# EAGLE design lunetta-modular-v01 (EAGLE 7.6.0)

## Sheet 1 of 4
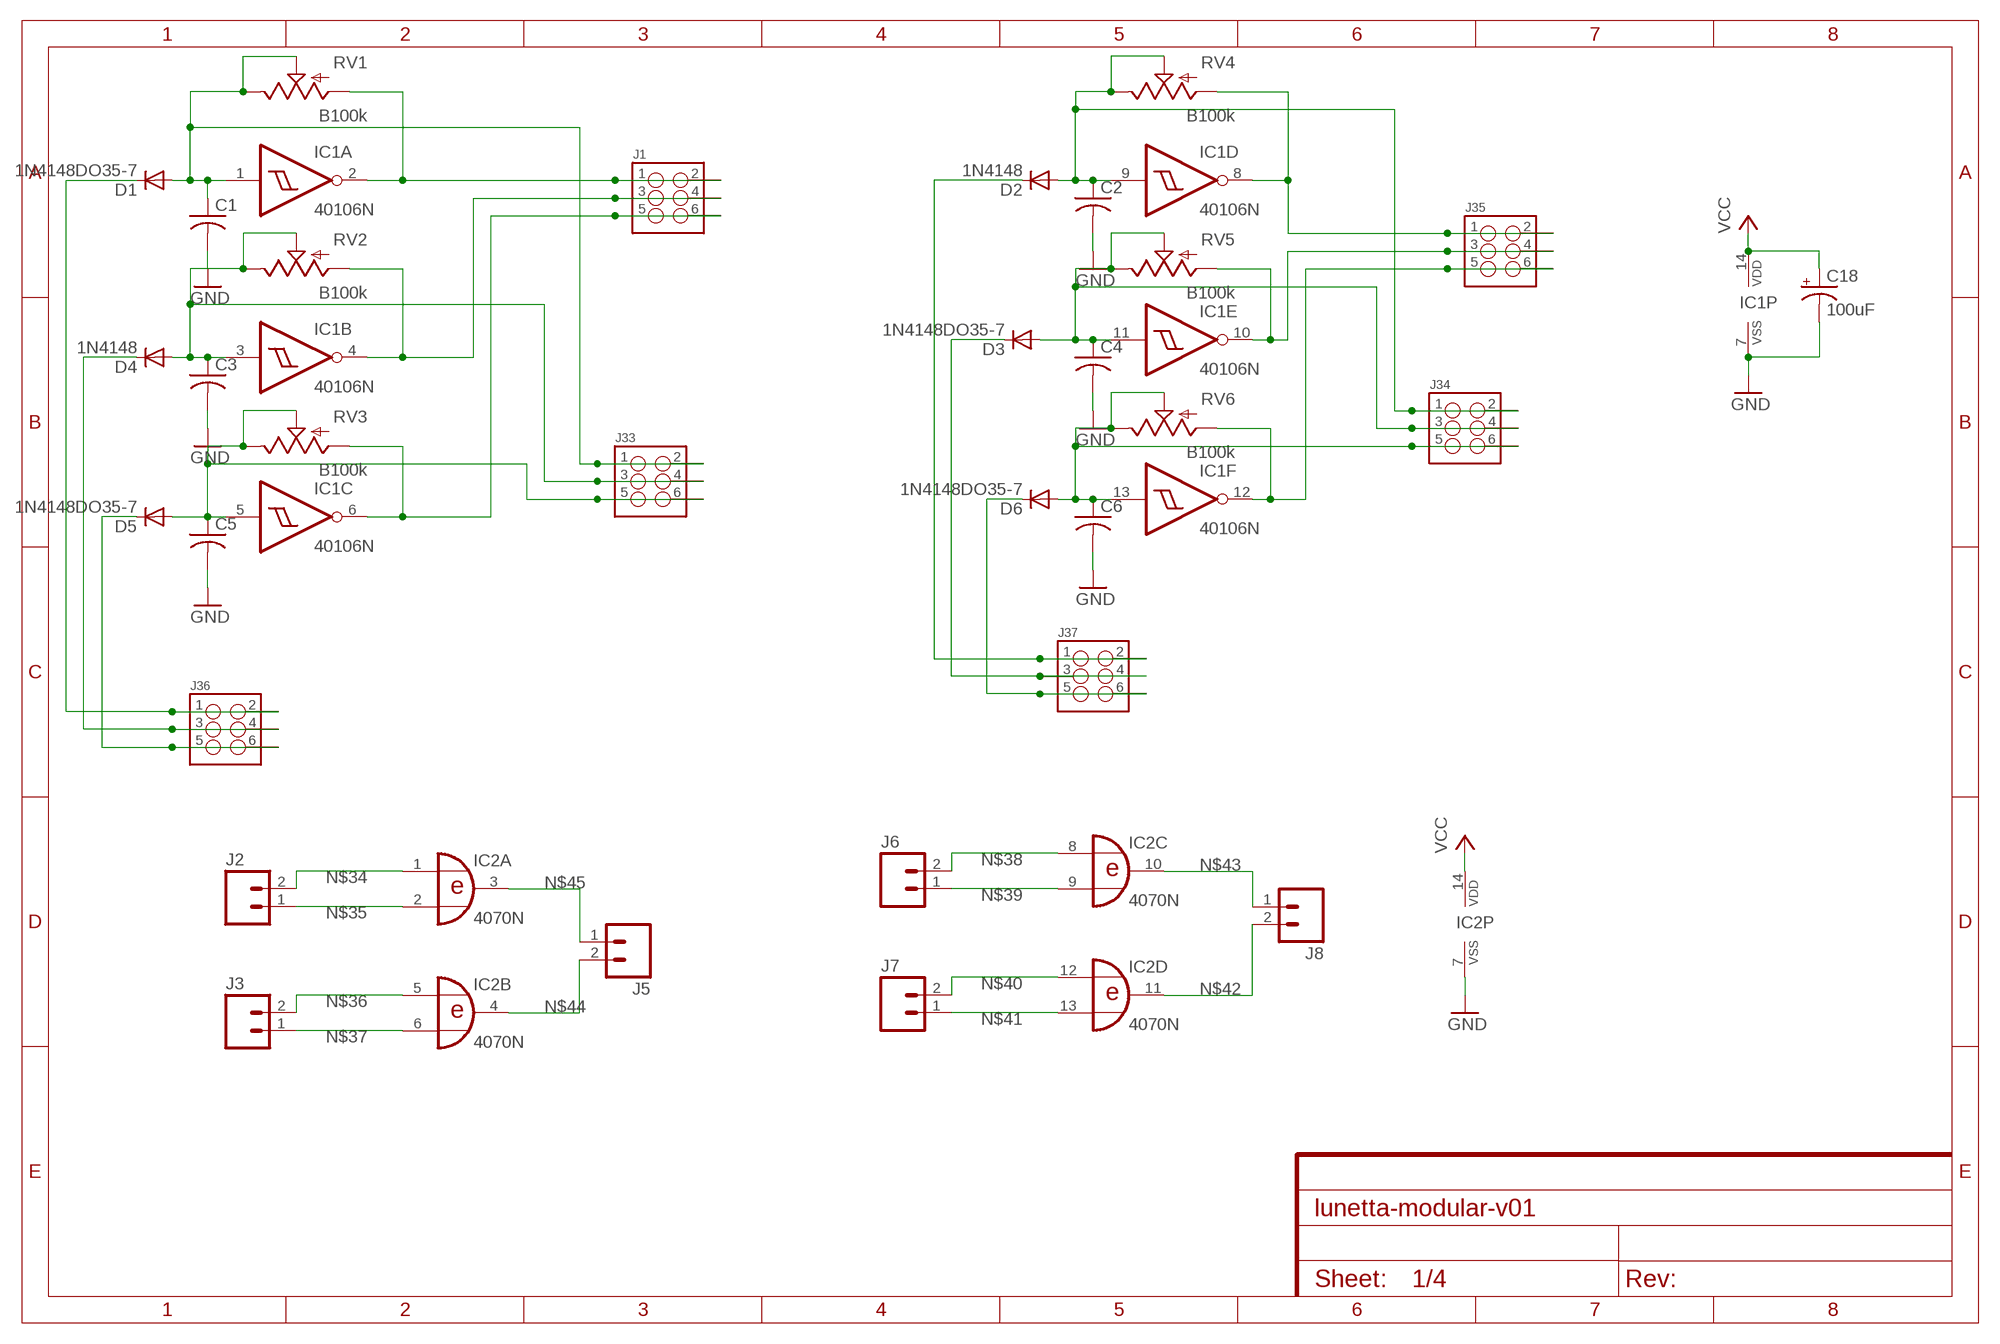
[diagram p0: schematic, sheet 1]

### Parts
C1  C-USC025_050-025X075_2GND  [C025_050-025X075]
C2  C-USC025_050-025X075_2GND  [C025_050-025X075]
C3  C-USC025_050-025X075_2GND  [C025_050-025X075]
C4  C-USC025_050-025X075_2GND  [C025_050-025X075]
C5  C-USC025_050-025X075_2GND  [C025_050-025X075]
C6  C-USC025_050-025X075_2GND  [C025_050-025X075]
C18  100uF  100UF-25V-20%(PTH)  [CPOL-RADIAL-100UF-25V]
D1  1N4148DO35-7  [DO35-7]
D2  1N4148  1N4148DO35-7  [DO35-7]
D3  1N4148DO35-7  [DO35-7]
D4  1N4148  1N4148DO35-7  [DO35-7]
D5  1N4148DO35-7  [DO35-7]
D6  1N4148DO35-7  [DO35-7]
IC1  40106N  [DIL14]
IC2  4070N  [DIL14]
J1  M03X22X3_SILK_MALE_PTH  [2X3]
J2  M02LOCK  [1X02_LOCK]
J3  M02LOCK  [1X02_LOCK]
J5  M02LOCK  [1X02_LOCK]
J6  M02LOCK  [1X02_LOCK]
J7  M02LOCK  [1X02_LOCK]
J8  M02LOCK  [1X02_LOCK]
J33  M03X22X3_SILK_MALE_PTH  [2X3]
J34  M03X22X3_SILK_MALE_PTH  [2X3]
J35  M03X22X3_SILK_MALE_PTH  [2X3]
J36  M03X22X3_SILK_MALE_PTH  [2X3]
J37  M03X22X3_SILK_MALE_PTH  [2X3]
RV1  B100k  POTELCON  [ALPS_POT_ELCON]
RV2  B100k  POTELCON  [ALPS_POT_ELCON]
RV3  B100k  POTELCON  [ALPS_POT_ELCON]
RV4  B100k  POTELCON  [ALPS_POT_ELCON]
RV5  B100k  POTELCON  [ALPS_POT_ELCON]
RV6  B100k  POTELCON  [ALPS_POT_ELCON]

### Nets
GND: C1.2 C1.3 C2.2 C2.3 C3.2 C3.3 C4.2 C4.3 C5.2 C5.3 C6.2 C6.3 C18.2(-) IC1.7(P:VSS) IC2.7(P:VSS) ; also sheet 2,3,4
N$1: D1.C J36.1 J36.2
N$2: D4.C J36.3 J36.4
N$3: D5.C J36.5 J36.6
N$4: D2.C J37.1 J37.2
N$5: D3.C J37.3 J37.4
N$6: D6.C J37.5 J37.6
N$19: IC1.8(D:O) J35.1 J35.2 RV4.P$3(A)
N$31: IC1.4(B:O) J1.3 J1.4 RV2.P$3(A)
N$32: IC1.10(E:O) J35.3 J35.4 RV5.P$3(A)
N$33: IC1.6(C:O) J1.5 J1.6 RV3.P$3(A)
N$34: IC2.1(A:I0) J2.2
N$35: IC2.2(A:I1) J2.1
N$36: IC2.5(B:I0) J3.2
N$37: IC2.6(B:I1) J3.1
N$38: IC2.8(C:I0) J6.2
N$39: IC2.9(C:I1) J6.1
N$40: IC2.12(D:I0) J7.2
N$41: IC2.13(D:I1) J7.1
N$42: IC2.11(D:O) J8.2
N$43: IC2.10(C:O) J8.1
N$44: IC2.4(B:O) J5.2
N$45: IC2.3(A:O) J5.1
N$89: IC1.12(F:O) J35.5 J35.6 RV6.P$3(A)
N$125: IC1.2(A:O) J1.1 J1.2 RV1.P$3(A)
N$127: C1.1 D1.A IC1.1(A:I) J33.1 J33.2 RV1.P$1(E) RV1.P$2(S)
N$131: C3.1 D4.A IC1.3(B:I) J33.3 J33.4 RV2.P$1(E) RV2.P$2(S)
N$144: C5.1 D5.A IC1.5(C:I) J33.5 J33.6 RV3.P$1(E) RV3.P$2(S)
N$145: C2.1 D2.A IC1.9(D:I) J34.1 J34.2 RV4.P$1(E) RV4.P$2(S)
N$146: C4.1 D3.A IC1.11(E:I) J34.3 J34.4 RV5.P$1(E) RV5.P$2(S)
N$147: C6.1 D6.A IC1.13(F:I) J34.5 J34.6 RV6.P$1(E) RV6.P$2(S)
VCC: C18.1(+) IC1.14(P:VDD) IC2.14(P:VDD) ; also sheet 2,3,4

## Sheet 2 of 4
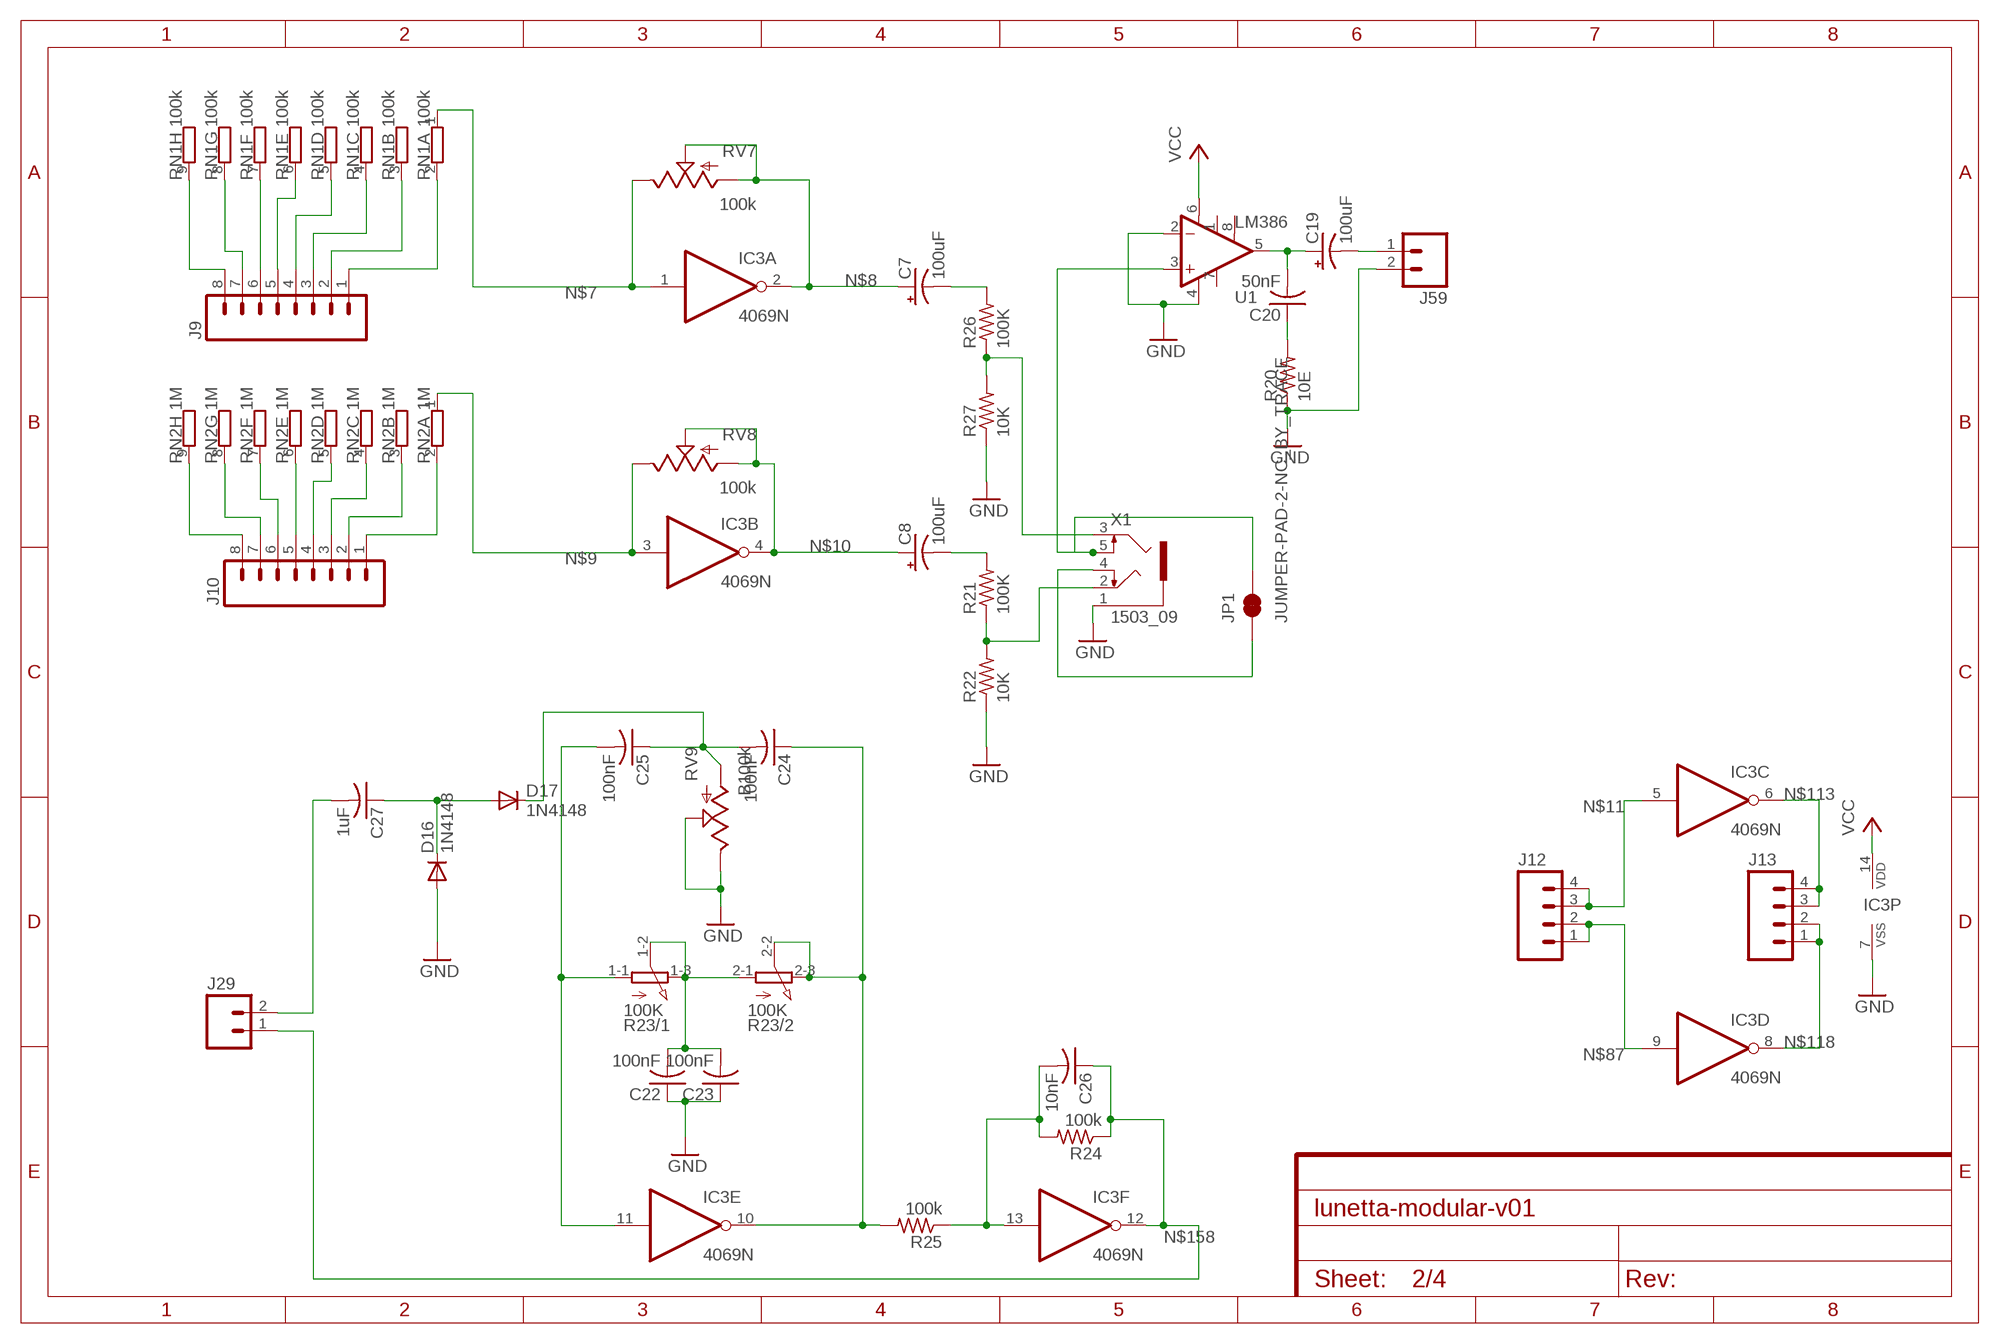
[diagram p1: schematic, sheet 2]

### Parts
C7  100uF  100UF-25V-20%(PTH)  [CPOL-RADIAL-100UF-25V]
C8  100uF  100UF-25V-20%(PTH)  [CPOL-RADIAL-100UF-25V]
C19  100uF  100UF-25V-20%(PTH)  [CPOL-RADIAL-100UF-25V]
C20  50nF  C-US025-025X050  [C025-025X050]
C22  100nF  C-US025-025X050  [C025-025X050]
C23  100nF  C-US025-025X050  [C025-025X050]
C24  100nF  C-US025-025X050  [C025-025X050]
C25  100nF  C-US025-025X050  [C025-025X050]
C26  10nF  C-US025-025X050  [C025-025X050]
C27  1uF  C-US025-025X050  [C025-025X050]
D16  1N4148  1N4148DO35-7  [DO35-7]
D17  1N4148  1N4148DO35-7  [DO35-7]
IC3  4069N  [DIL14]
J9  M08LOCK  [1X08_LOCK]
J10  M08LOCK  [1X08_LOCK]
J12  M042X2  [2X2]
J13  M042X2  [2X2]
J29  M02LOCK  [1X02_LOCK]
J59  M02LOCK  [1X02_LOCK]
JP1  JUMPER-PAD-2-NC_BY_TRACE  [PAD-JUMPER-2-NC_BY_TRACE_YES_SILK]
R20  10E  R-US_0207/10  [0207/10]
R21  100K  R-US_0207/10  [0207/10]
R22  10K  R-US_0207/10  [0207/10]
R23  100K  3RP/1610G  [3RP/1610G]
R24  100k  R-US_0207/10  [0207/10]
R25  100k  R-US_0207/10  [0207/10]
R26  100K  R-US_0207/10  [0207/10]
R27  10K  R-US_0207/10  [0207/10]
RN1  100k  GE08R  [SIL9]
RN2  1M  GE08R  [SIL9]
RV7  100k  POTELCON  [ALPS_POT_ELCON]
RV8  100k  POTELCON  [ALPS_POT_ELCON]
RV9  B100k  POTELCON  [ALPS_POT_ELCON]
U1  LM386  [DIP08]
X1  1503_09  [1503_09]

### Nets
GND: C22.1 C23.1 D16.A IC3.7(P:VSS) J59.2 R20.1 R22.1 R27.1 RV9.P$1(E) RV9.P$2(S) U1.2(-IN) U1.4(V-) X1.1 ; also sheet 1,3,4
N$7: IC3.1(A:I) RN1.1 RV7.P$1(E)
N$8: C7.1(+) IC3.2(A:O) RV7.P$2(S) RV7.P$3(A)
N$9: IC3.3(B:I) RN2.1 RV8.P$1(E)
N$10: C8.1(+) IC3.4(B:O) RV8.P$2(S) RV8.P$3(A)
N$11: IC3.5(C:I) J12.3 J12.4
N$13: JP1.1 X1.4
N$15: C20.1 R20.2
N$16: C19.1(+) C20.2 U1.5(OUT)
N$28: C8.2(-) R21.2
N$87: IC3.9(D:I) J12.1 J12.2
N$88: R26.1 R27.2 X1.3
N$90: C27.2 J29.2
N$92: C26.2 IC3.13(F:I) R24.2 R25.1
N$95: J10.8 RN2.9
N$96: J10.7 RN2.8
N$99: J10.6 RN2.7
N$100: J10.5 RN2.6
N$101: J10.4 RN2.5
N$102: J10.3 RN2.4
N$103: J10.2 RN2.3
N$104: J10.1 RN2.2
N$105: J9.8 RN1.9
N$106: J9.7 RN1.8
N$107: J9.6 RN1.7
N$108: J9.5 RN1.6
N$109: J9.4 RN1.5
N$110: J9.3 RN1.4
N$111: J9.2 RN1.3
N$112: J9.1 RN1.2
N$113: IC3.6(C:O) J13.3 J13.4
N$115: C7.2(-) R26.2
N$118: IC3.8(D:O) J13.1 J13.2
N$130: C19.2(-) J59.1
N$148: R21.1 R22.2 X1.2
N$151: JP1.2 U1.3(+IN) X1.5
N$153: C27.1 D16.C D17.A
N$154: C24.2 C25.1 D17.C RV9.P$3(A)
N$155: C22.2 C23.2 R23.1-2(/1:S) R23.1-3(/1:E) R23.2-1(/2:A)
N$156: C24.1 IC3.10(E:O) R23.2-2(/2:S) R23.2-3(/2:E) R25.2
N$157: C25.2 IC3.11(E:I) R23.1-1(/1:A)
N$158: C26.1 IC3.12(F:O) J29.1 R24.1
VCC: IC3.14(P:VDD) U1.6(V+) ; also sheet 1,3,4
Unconnected: U1.1(GAIN) U1.7(BP) U1.8(GAIN)

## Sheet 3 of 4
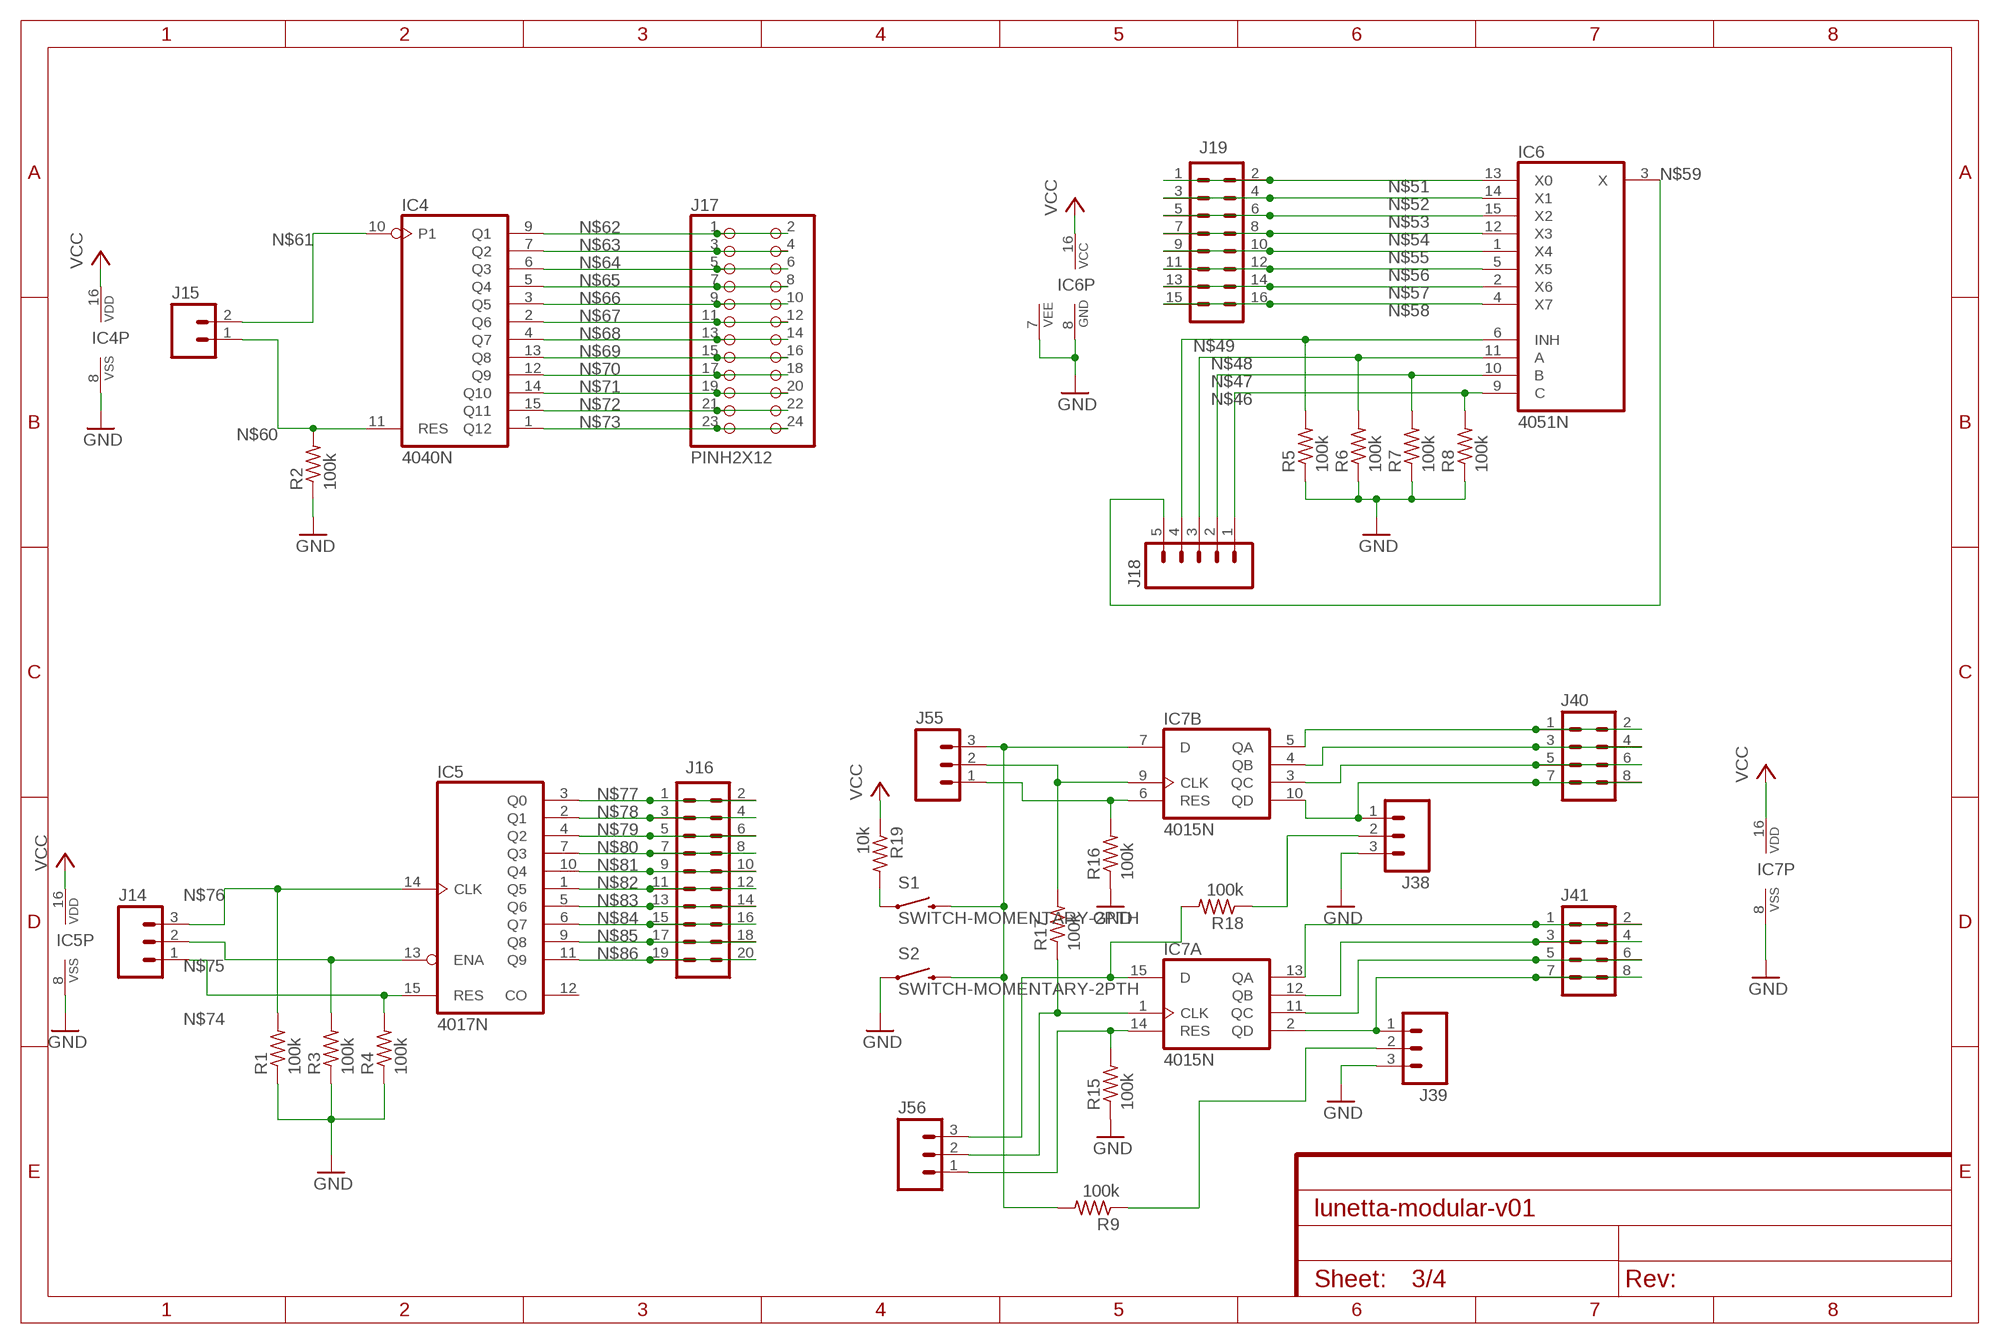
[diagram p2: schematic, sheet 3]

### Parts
IC4  4040N  [DIL16]
IC5  4017N  [DIL16]
IC6  4051N  [DIL16]
IC7  4015N  [DIL16]
J14  M03LOCK  [1X03_LOCK]
J15  M02PTH  [1X02]
J16  M10X2  [2X10]
J17  PINH2X12  [2X12]
J18  M05LOCK  [1X05_LOCK]
J19  M08X2  [2X8]
J38  M03LOCK  [1X03_LOCK]
J39  M03LOCK  [1X03_LOCK]
J40  M04X2  [2X4]
J41  M04X2  [2X4]
J55  M03LOCK  [1X03_LOCK]
J56  M03LOCK  [1X03_LOCK]
R1  100k  R-US_0207/10  [0207/10]
R2  100k  R-US_0207/10  [0207/10]
R3  100k  R-US_0207/10  [0207/10]
R4  100k  R-US_0207/10  [0207/10]
R5  100k  R-US_0207/10  [0207/10]
R6  100k  R-US_0207/10  [0207/10]
R7  100k  R-US_0207/10  [0207/10]
R8  100k  R-US_0207/10  [0207/10]
R9  100k  R-US_0207/10  [0207/10]
R15  100k  R-US_0207/10  [0207/10]
R16  100k  R-US_0207/10  [0207/10]
R17  100k  R-US_0207/10  [0207/10]
R18  100k  R-US_0207/10  [0207/10]
R19  10k  R-US_0207/10  [0207/10]
S1  SWITCH-MOMENTARY-2PTH  [TACTILE-PTH]
S2  SWITCH-MOMENTARY-2PTH  [TACTILE-PTH]

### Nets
GND: IC4.8(VSS) IC5.8(VSS) IC6.7(VEE) IC6.8(GND) IC7.8(P:VSS) J38.3 J39.3 R1.1 R2.1 R3.1 R4.1 R5.1 R6.1 R7.1 R8.1 R15.1 R16.1 S2.1 ; also sheet 1,2,4
N$12: J39.2 R9.1
N$46: IC6.9(C) J18.1 R8.2
N$47: IC6.10(B) J18.2 R7.2
N$48: IC6.11(A) J18.3 R6.2
N$49: IC6.6(INH) J18.4 R5.2
N$51: IC6.13(X0) J19.1 J19.2
N$52: IC6.14(X1) J19.3 J19.4
N$53: IC6.15(X2) J19.5 J19.6
N$54: IC6.12(X3) J19.7 J19.8
N$55: IC6.1(X4) J19.9 J19.10
N$56: IC6.5(X5) J19.11 J19.12
N$57: IC6.2(X6) J19.13 J19.14
N$58: IC6.4(X7) J19.15 J19.16
N$59: IC6.3(X) J18.5
N$60: IC4.11(RES) J15.1 R2.2
N$61: IC4.10(P1) J15.2
N$62: IC4.9(Q1) J17.1 J17.2
N$63: IC4.7(Q2) J17.3 J17.4
N$64: IC4.6(Q3) J17.5 J17.6
N$65: IC4.5(Q4) J17.7 J17.8
N$66: IC4.3(Q5) J17.9 J17.10
N$67: IC4.2(Q6) J17.11 J17.12
N$68: IC4.4(Q7) J17.13 J17.14
N$69: IC4.13(Q8) J17.15 J17.16
N$70: IC4.12(Q9) J17.17 J17.18
N$71: IC4.14(Q10) J17.19 J17.20
N$72: IC4.15(Q11) J17.21 J17.22
N$73: IC4.1(Q12) J17.23 J17.24
N$74: IC5.15(RES) J14.1 R4.2
N$75: IC5.13(ENA) J14.2 R3.2
N$76: IC5.14(CLK) J14.3 R1.2
N$77: IC5.3(Q0) J16.1 J16.2
N$78: IC5.2(Q1) J16.3 J16.4
N$79: IC5.4(Q2) J16.5 J16.6
N$80: IC5.7(Q3) J16.7 J16.8
N$81: IC5.10(Q4) J16.9 J16.10
N$82: IC5.1(Q5) J16.11 J16.12
N$83: IC5.5(Q6) J16.13 J16.14
N$84: IC5.6(Q7) J16.15 J16.16
N$85: IC5.9(Q8) J16.17 J16.18
N$86: IC5.11(Q9) J16.19 J16.20
N$97: IC7.14(A:RES) J56.1 R15.2
N$98: IC7.6(B:RES) J55.1 R16.2
N$124: IC7.9(B:CLK) J55.2 R17.2
N$126: IC7.1(A:CLK) J56.2 R17.1
N$132: IC7.10(B:QD) J38.1 J40.7 J40.8
N$133: IC7.15(A:D) J56.3 R18.2
N$134: J38.2 R18.1
N$135: IC7.2(A:QD) J39.1 J41.7 J41.8
N$136: IC7.7(B:D) J55.3 R9.2 S1.3 S2.3
N$137: R19.2 S1.1
N$138: IC7.11(A:QC) J41.5 J41.6
N$139: IC7.12(A:QB) J41.3 J41.4
N$140: IC7.13(A:QA) J41.1 J41.2
N$141: IC7.3(B:QC) J40.5 J40.6
N$142: IC7.4(B:QB) J40.3 J40.4
N$143: IC7.5(B:QA) J40.1 J40.2
VCC: IC4.16(VDD) IC5.16(VDD) IC6.16(VCC) IC7.16(P:VDD) R19.1 ; also sheet 1,2,4
Unconnected: IC5.12(CO)

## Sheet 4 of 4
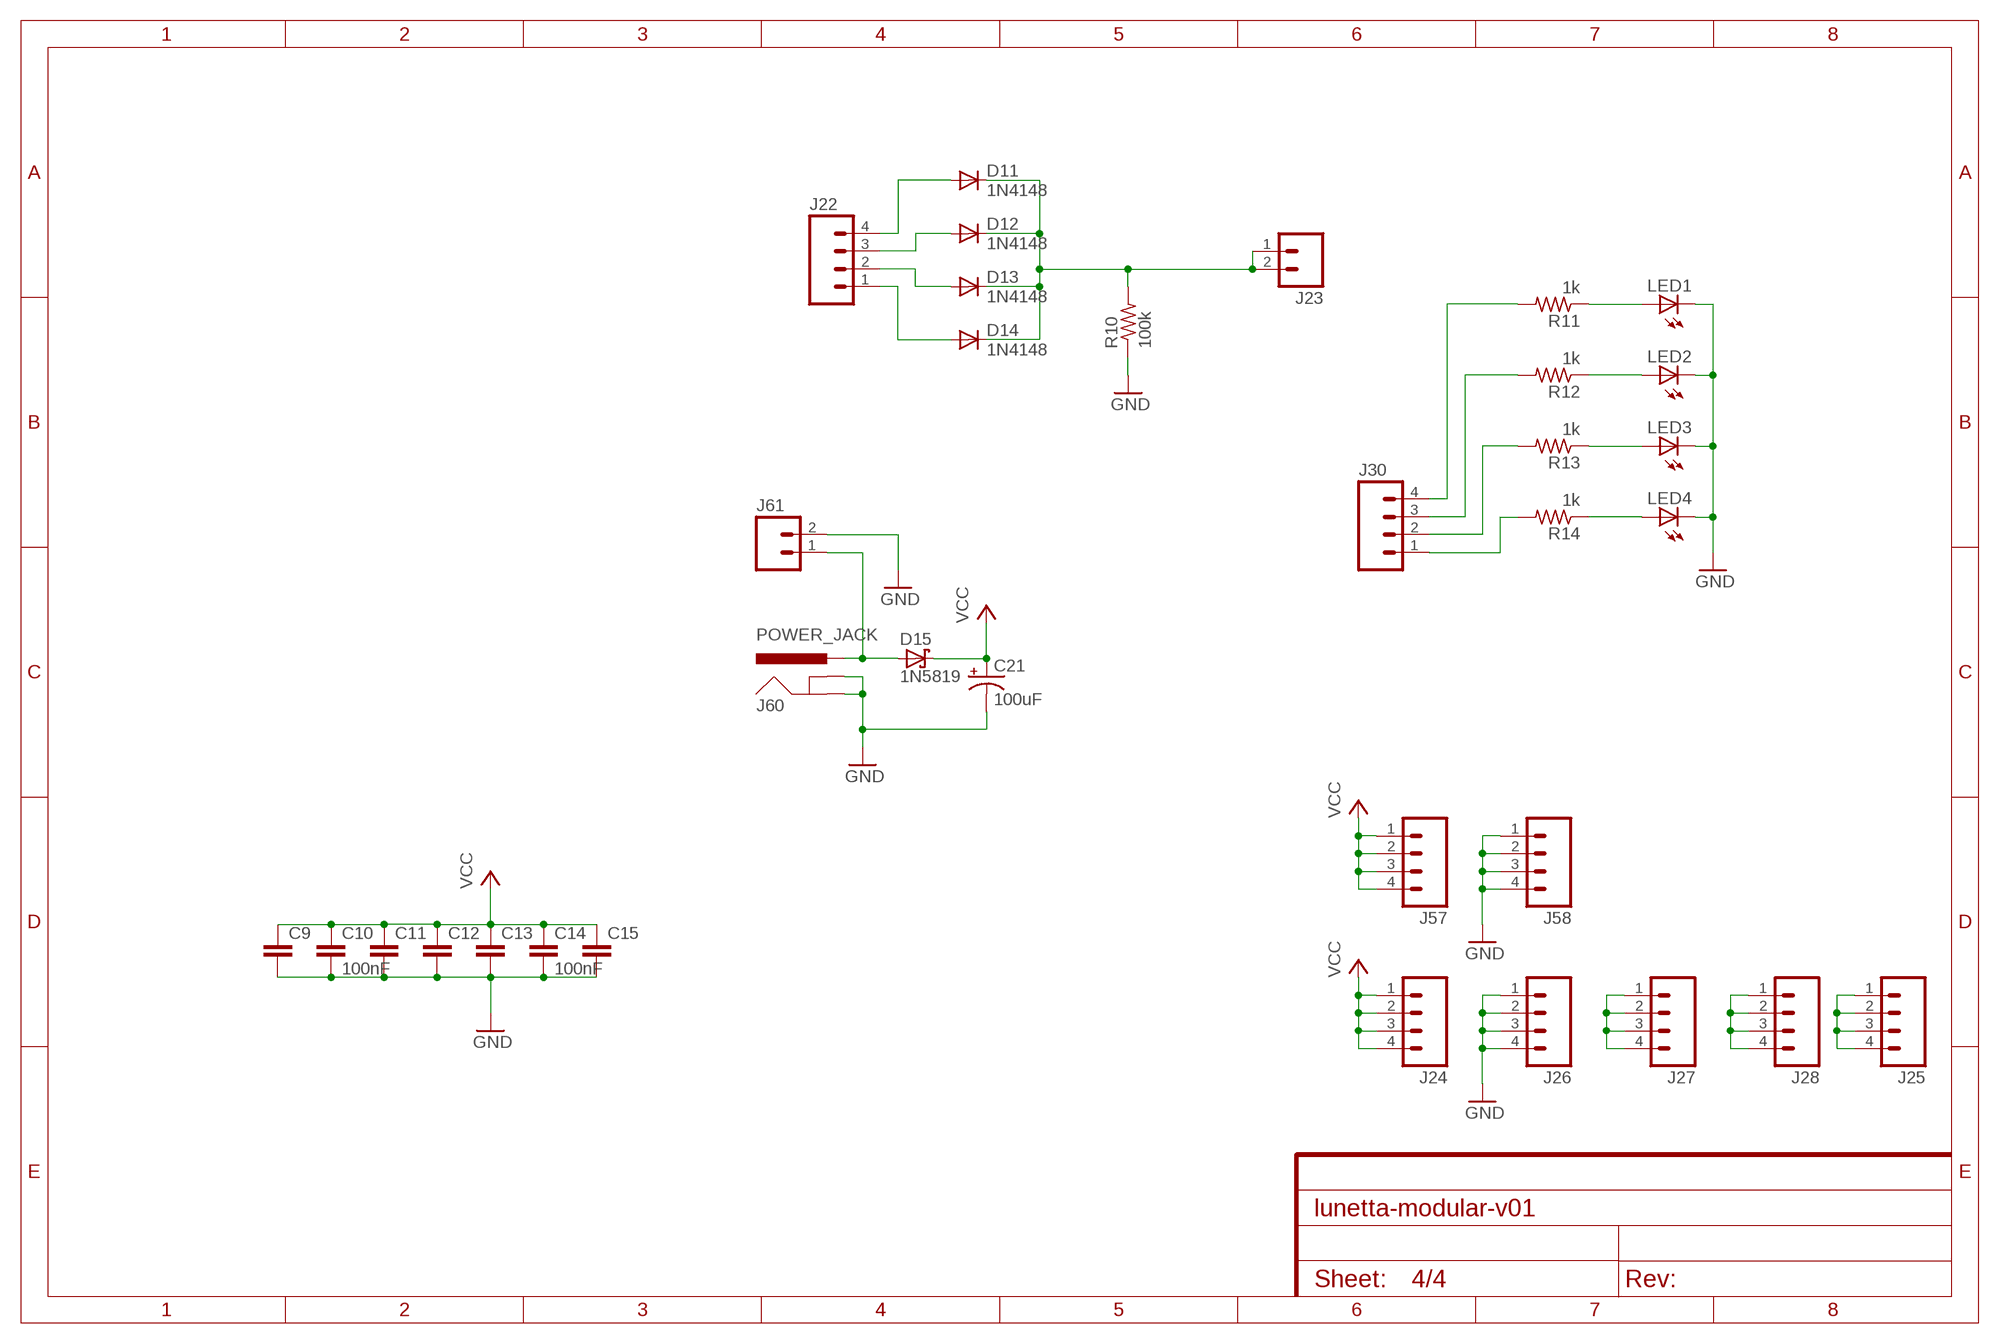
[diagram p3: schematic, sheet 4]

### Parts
C9  CAPPTH2  [CAP-PTH-SMALL2]
C10  100nF  CAPPTH2  [CAP-PTH-SMALL2]
C11  CAPPTH2  [CAP-PTH-SMALL2]
C12  CAPPTH2  [CAP-PTH-SMALL2]
C13  CAPPTH2  [CAP-PTH-SMALL2]
C14  100nF  CAPPTH2  [CAP-PTH-SMALL2]
C15  CAPPTH2  [CAP-PTH-SMALL2]
C21  100uF  100UF-25V-20%(PTH)  [CPOL-RADIAL-100UF-25V]
D11  1N4148  1N4148DO35-7  [DO35-7]
D12  1N4148  1N4148DO35-7  [DO35-7]
D13  1N4148  1N4148DO35-7  [DO35-7]
D14  1N4148  1N4148DO35-7  [DO35-7]
D15  1N5819  1N5819-B  [DO41-7.6]
J22  M04LOCK  [1X04_LOCK]
J23  M02PTH  [1X02]
J24  M04LOCK  [1X04_LOCK]
J25  M04LOCK  [1X04_LOCK]
J26  M04LOCK  [1X04_LOCK]
J27  M04LOCK  [1X04_LOCK]
J28  M04LOCK  [1X04_LOCK]
J30  M04LOCK  [1X04_LOCK]
J57  M04LOCK  [1X04_LOCK]
J58  M04LOCK  [1X04_LOCK]
J60  POWER_JACK  POWER_JACKPTH  [POWER_JACK_PTH]
J61  M02PTH  [1X02]
LED1  LED3MM  [LED3MM]
LED2  LED3MM  [LED3MM]
LED3  LED3MM  [LED3MM]
LED4  LED3MM  [LED3MM]
R10  100k  R-US_0207/10  [0207/10]
R11  1k  R-US_0207/10  [0207/10]
R12  1k  R-US_0207/10  [0207/10]
R13  1k  R-US_0207/10  [0207/10]
R14  1k  R-US_0207/10  [0207/10]

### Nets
GND: C9.2 C10.2 C11.2 C12.2 C13.2 C14.2 C15.2 C21.2(-) J26.1 J26.2 J26.3 J26.4 J58.1 J58.2 J58.3 J58.4 J60.GND J60.GNDBREAK J61.2 LED1.K(C) LED2.K(C) LED3.K(C) LED4.K(C) R10.1 ; also sheet 1,2,3
N$17: D15.A J60.PWR J61.1
N$20: LED4.A R14.1
N$23: J27.1 J27.2 J27.3 J27.4
N$24: J28.1 J28.2 J28.3 J28.4
N$25: LED3.A R13.1
N$26: LED2.A R12.1
N$27: LED1.A R11.1
N$30: J30.1 R14.2
N$91: J30.2 R13.2
N$93: J30.3 R12.2
N$94: J30.4 R11.2
N$116: D11.A J22.4
N$117: D12.A J22.3
N$121: D13.A J22.2
N$122: D14.A J22.1
N$123: D11.C D12.C D13.C D14.C J23.1 J23.2 R10.2
N$128: J25.1 J25.2 J25.3 J25.4
VCC: C9.1 C10.1 C11.1 C12.1 C13.1 C14.1 C15.1 C21.1(+) D15.C J24.1 J24.2 J24.3 J24.4 J57.1 J57.2 J57.3 J57.4 ; also sheet 1,2,3

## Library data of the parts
C1-C6 C20 C22-C27 = adafruit:C-US: CAPACITOR, American symbol
C7 C8 C18 C19 C21 = SparkFun-Capacitors:100UF-25V-20%(PTH): CAP-08439; PROD_ID: CAP-08439
C9-C15 = SparkFun-Capacitors:CAP: Capacitor
D1-D6 D11-D14 D16 D17 = diode:1N4148: DIODE
D15 = diode:1N581*: 1.0A SCHOTTKY BARRIER RECTIFIER
IC1 = 40xx:40106: Hex SCHMITT TRIGGER
IC2 = 40xx:4070: Quad 2-input XOR
IC3 = 40xx:4069: Hex INVERTER
IC4 = 40xx:4040: 12-stage binary/ripple COUNTER
IC5 = 40xx:4017: COUNTER/DIVIDER
IC6 = 40xx:4051: 8-channel ANALOG MULTIPLEXER
IC7 = 40xx:4015: Dual 4-bit static SHIFT REGISTER
J1 J33-J37 = SparkFun-Connectors:M03X2: 2x3 .1" header. Shrouded, with keying- CONN-10681 SMT- CONN-11415 Pogo pins- HW-11044; PROD_ID: CONN-09701
J2 J3 J5-J8 J15 J23 J29 J59 J61 = SparkFun-Connectors:M02: Standard 2-pin 0.1" header. Use with
J9 J10 = SparkFun-Connectors:M08: Header 8 Standard 8-pin 0.1" header. Use with straight break away headers (SKU : PRT-00116), right angle break away headers (PRT-00553), swiss pins (PRT-00743), machine pins (PRT-00117), and female headers (PRT-00115).
J12 J13 = SparkFun-Connectors:M04: Header 4 Standard 4-pin 0.1" header. Use with straight break away headers (SKU : PRT-00116), right angle break away headers (PRT-00553), swiss pins (PRT-00743), machine pins (PRT-00117), and female headers (PRT-00115). Molex polarized connector foot print use with SKU : PRT-08231 with associated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
J14 J38 J39 J55 J56 = SparkFun-Connectors:M03: Header 3 Standard 3-pin 0.1" header. Use with straight break away headers (SKU : PRT-00116), right angle break away headers (PRT-00553), swiss pins (PRT-00743), machine pins (PRT-00117), and female headers (PRT-00115). Molex polarized connector foot print use with SKU : PRT-08232 with associated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
J16 = SparkFun-Connectors:M10X2: This was SPECIALLY designed to be used with our Graphic LCD Backpack. Be sure you want to use this! It is not only staggered on each line of header holes, but IT IS ALSO offset of the center point of the top and bottom lines by 5 mil. This causes the headers to lock into place on the "standard"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
J17 = SparkFun-Connectors:PINH2X12
J18 = SparkFun-Connectors:M05: Header 5 Standard 5-pin 0.1" header. Use with straight break away headers (SKU : PRT-00116), right angle break away headers (PRT-00553), swiss pins (PRT-00743), machine pins (PRT-00117), and female headers (PRT-00115). Molex polarized connector foot print use with SKU : PRT-08230 with associated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
J19 = SparkFun-Connectors:M08X2: .1" headers, two rows of 8 each
J22 J24-J28 J30 J57 J58 = SparkFun-Connectors:M04: Header 4 Standard 4-pin 0.1" header. Use with straight break away headers (SKU : PRT-00116), right angle break away headers (PRT-00553), swiss pins (PRT-00743), machine pins (PRT-00117), and female headers (PRT-00115). Molex polarized connector foot print use with SKU : PRT-08231 with associated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; PROD_ID: CONN-09696
J40 J41 = SparkFun-Connectors:M04X2: .1" header, two rows of four.
J60 = SparkFun-Connectors:POWER_JACK: Power Jack This is the standard 5.5mm barrel jack for power. The PTH is the most common, proven, reliable, footprint. The Slot footprint only works if the mill layer is transmitted to the PCB fab house so be warned. Mating wall wart : TOL-00298 (and others); PROD_ID: CONN-08197
JP1 = SparkFun-Passives:JUMPER-PAD-2-NC_BY_TRACE
LED1-LED4 = adafruit:LED: LED
R1-R22 R24-R27 = adafruit:R-US_: RESISTOR, American symbol
R23 = pot:3RP/1610G: 16mm Potentiometer two level Source: http://www.alphapotentiometers.net/html/16mm_pot_2.html
RN1 RN2 = resistor-sil:GE08R: SIL RESISTOR; OC_FARNELL: unknown; OC_NEWARK: unknown
RV1-RV9 = SparkFun-Electromechanical:POT
S1 S2 = SparkFun-Electromechanical:SWITCH-MOMENTARY-2: Various NO switches- pushbuttons, reed, etc; PROD_ID: SWCH-08441
U1 = SparkFun-AnalogIC:LM386: low voltage audio power amplifier
X1 = con-lumberg:1503_09: Jack connectors according to JISC 6560, 3.5 mm Klinkeneinbaukupplung nach JISC 6560, 3,5 mm, 3-polig/ stereo, abgewinkelte Ausführung, mit 2 Öffnern und Lötaugen, für Leiterplatten Rückseitenmontage Source: http://www.lumberg.com/Produkte/PDFs/1503_09.pdf; OC_FARNELL: 1243244; OC_NEWARK: unknown

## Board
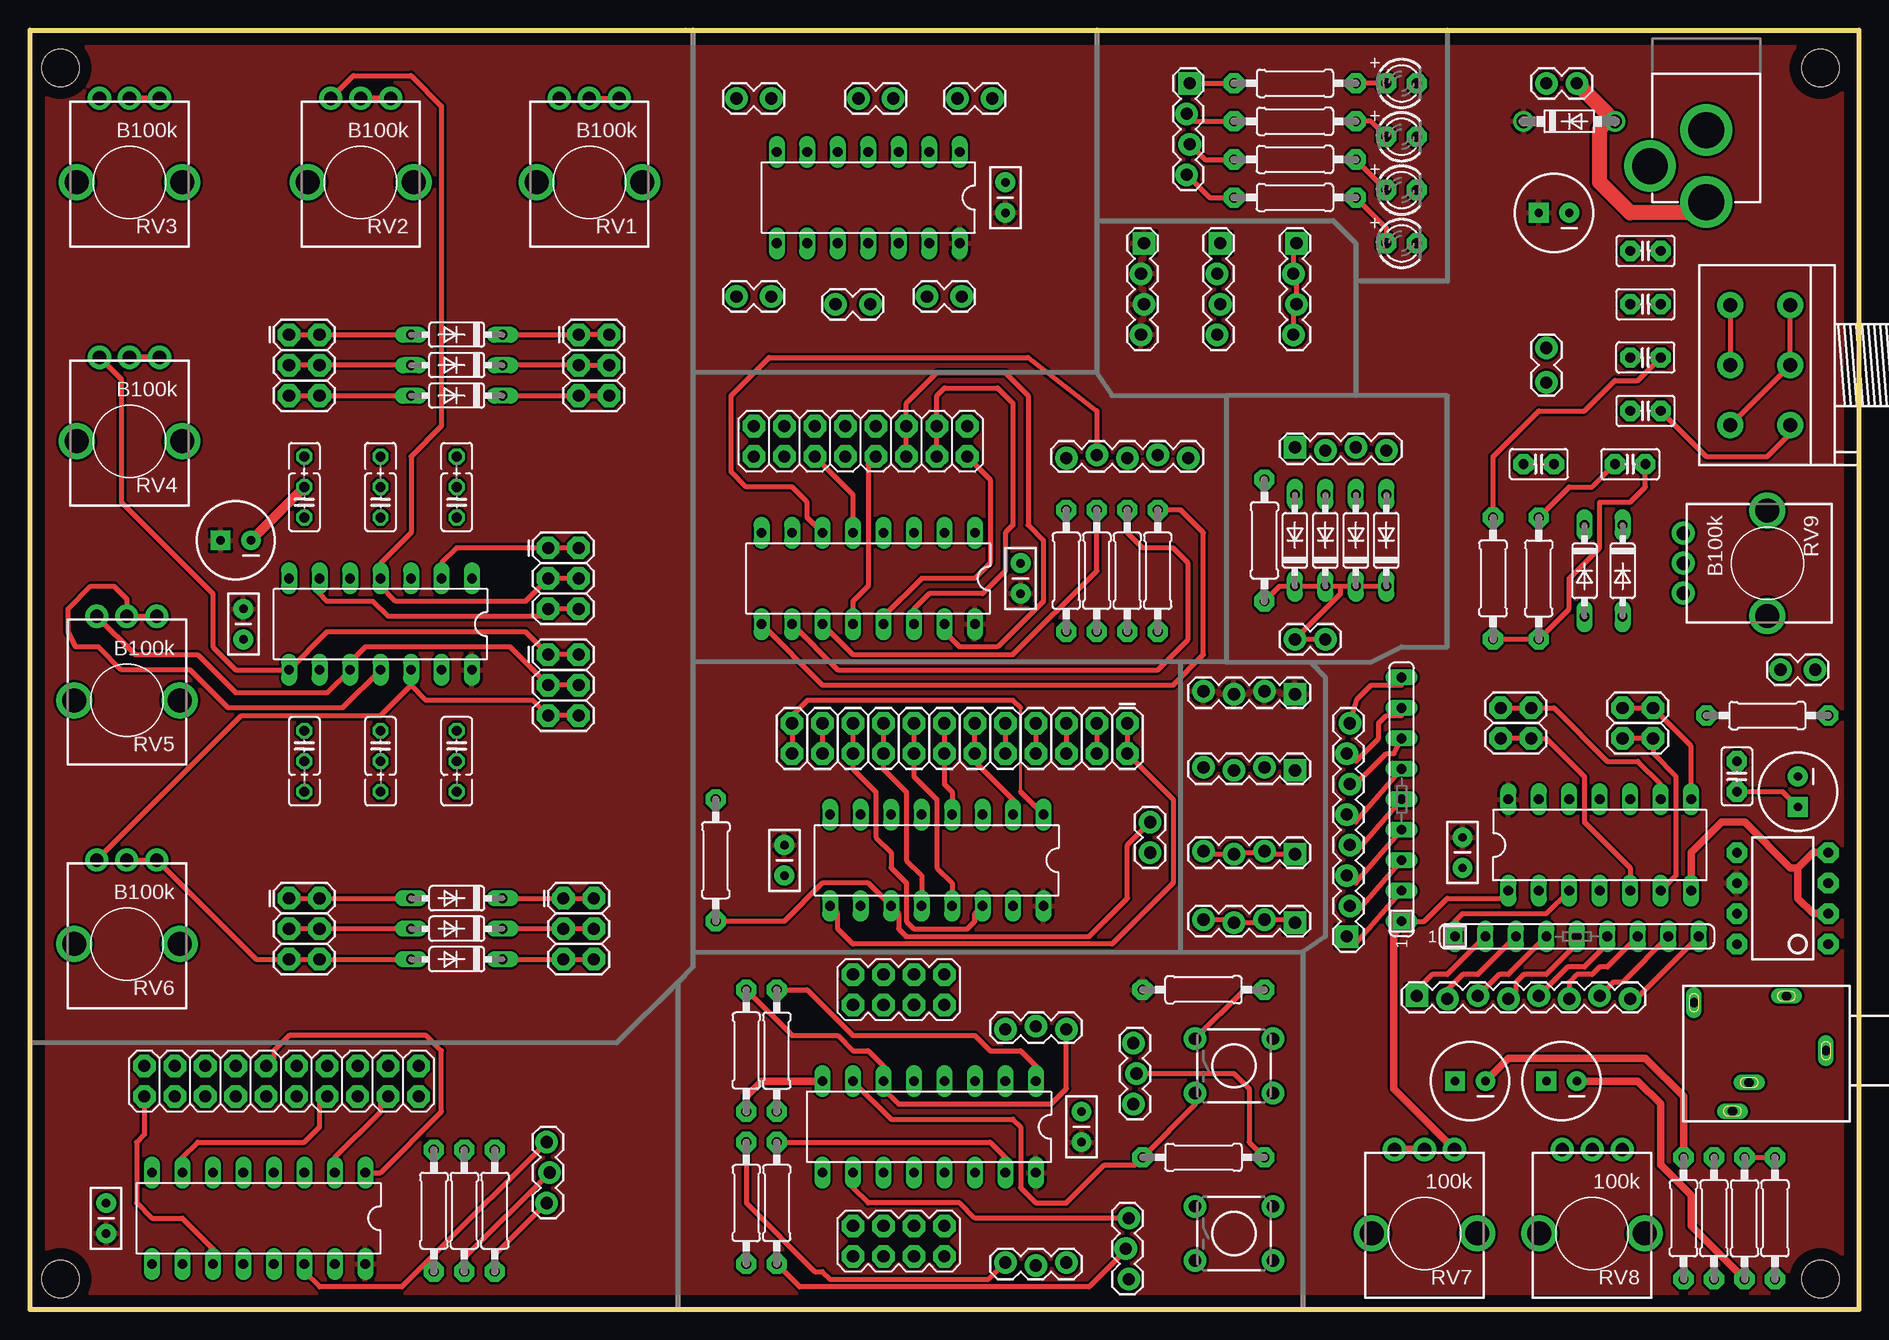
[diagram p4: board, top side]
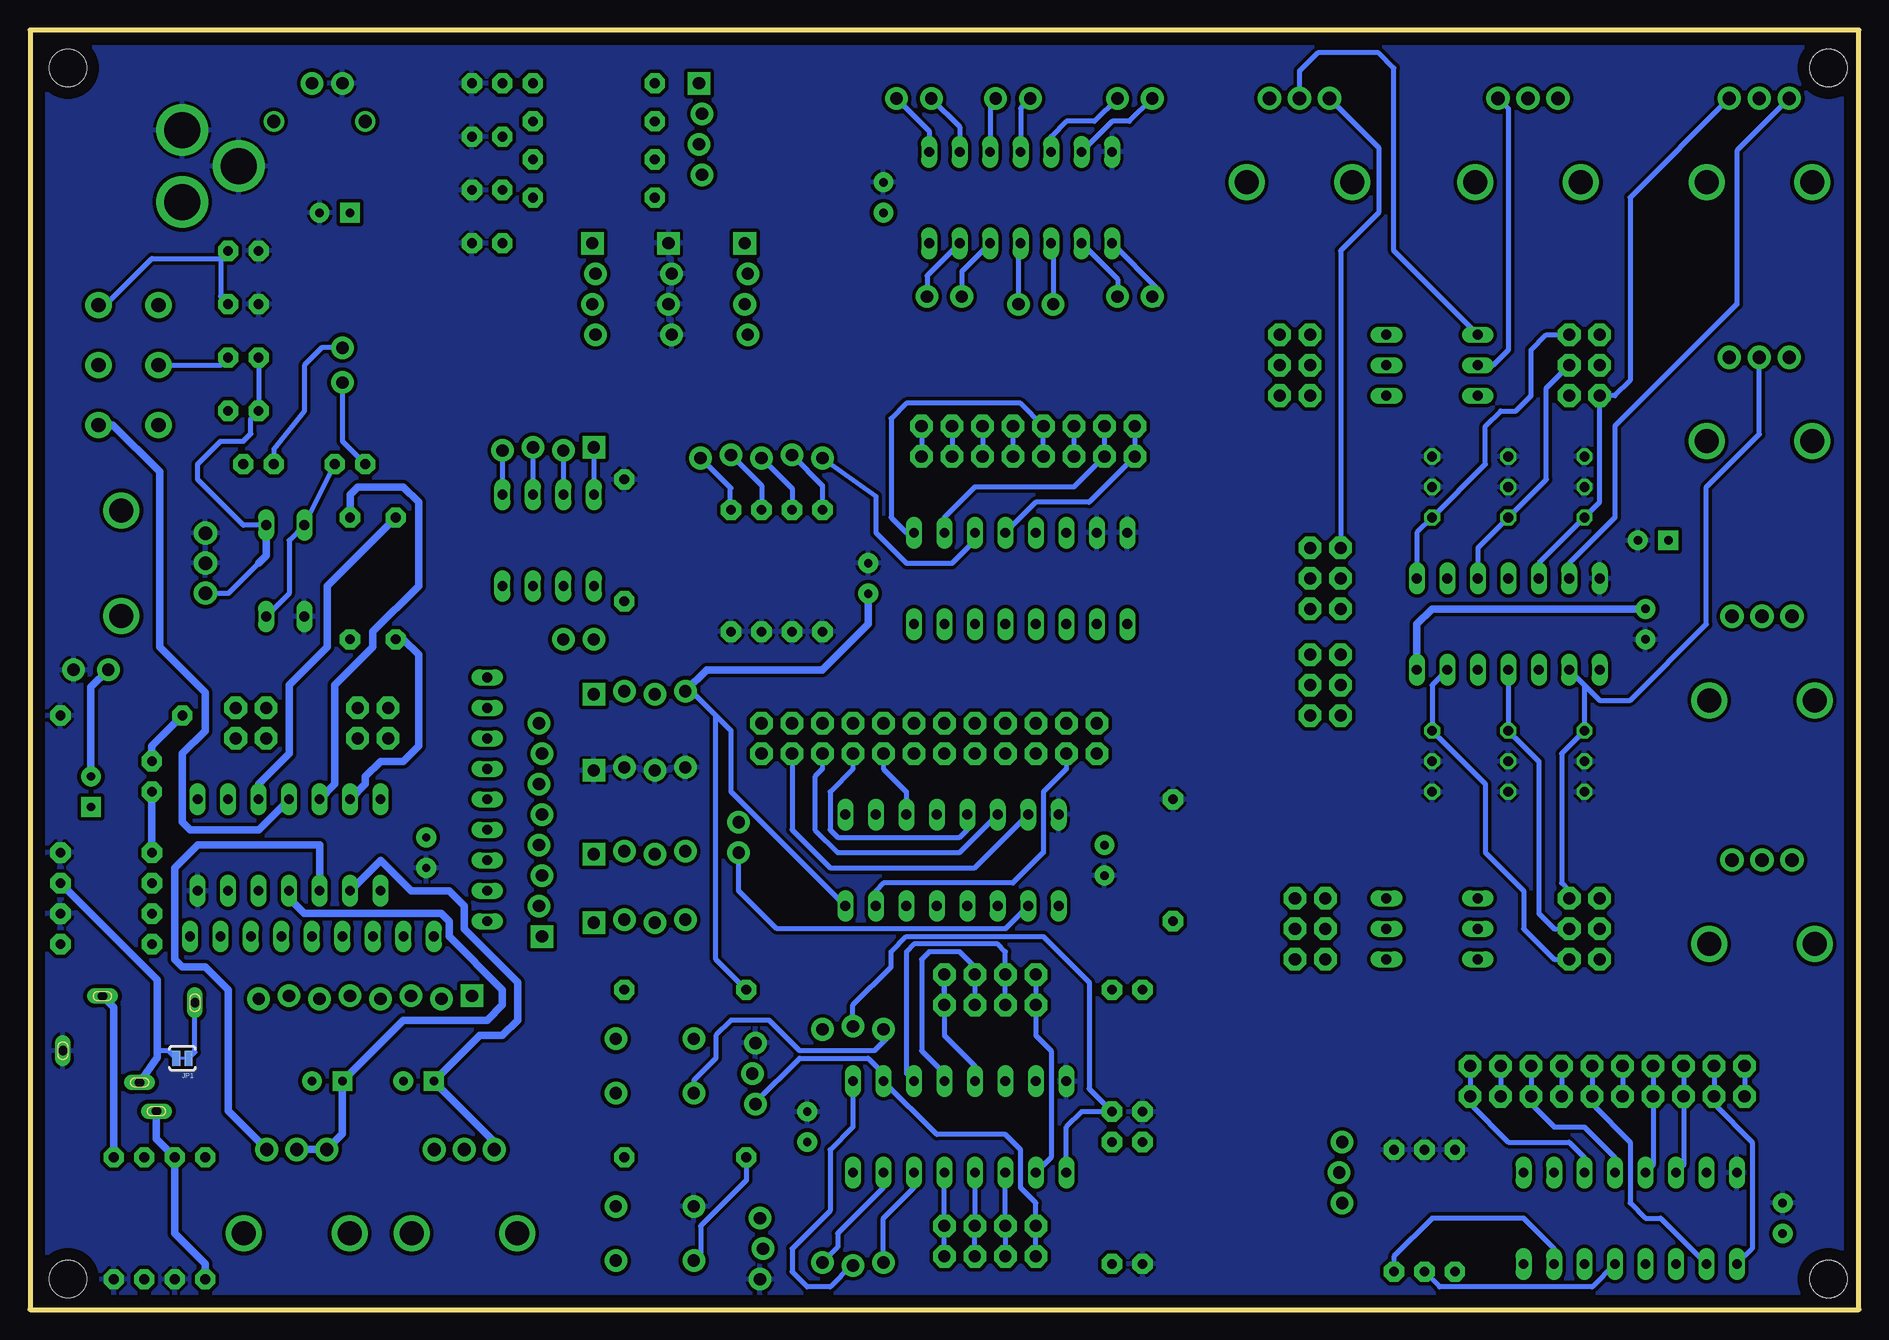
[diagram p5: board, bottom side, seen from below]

Size 152.4 x 106.68 mm. Coordinates in mm from the lower left corner, seen from the top.
Outline: 0,0 0,106.68 152.4,106.68 152.4,0 0,0
Copper layers (1*16): Top 0.035mm / dielectric 1.5mm / Bottom 0.035mm
Design rules "default": minimum track width 10mil, minimum drill 24mil, track to track 8mil, track to pad 8mil, pad to pad 8mil, via to via 8mil, smd to smd 8mil, copper to edge 40mil, drill to drill 8mil, minimum pad ring 10mil, minimum via ring 8mil, stop-mask expansion 4mil, vias tented up to drill 0mil, thermal gap 10mil
Holes 3.1 mm at 2.54,103.5 2.54,2.54 149.22,103.5 149.22,2.54

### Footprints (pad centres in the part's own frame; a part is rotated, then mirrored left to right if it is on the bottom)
C025_050-025X075 = drill 0.813 octagon: 1 -1.27,0; 2 1.27,0; 3 3.81,0
CPOL-RADIAL-100UF-25V = drill 0.7 pad 1.651 square: 1 1.27,0 | drill 0.7 pad 1.651: 2 -1.27,0
CAP-PTH-SMALL2 = drill 0.7 pad 1.651: 1 0,0; 2 2.54,0
C025-025X050 = drill 0.813 pad 1.676 octagon: 1 -1.27,0; 2 1.27,0
DO35-7 = drill 0.813 long: A 3.81,0; C -3.81,0
DO41-7.6 = drill 1.1 pad 1.7: A 3.81,0; C -3.81,0
DIL14 = drill 0.813 long: 1 -7.62,-3.81; 2 -5.08,-3.81; 3 -2.54,-3.81; 4 0,-3.81; 5 2.54,-3.81; 6 5.08,-3.81; 7 7.62,-3.81; 8 7.62,3.81; 9 5.08,3.81; 10 2.54,3.81; 11 0,3.81; 12 -2.54,3.81; 13 -5.08,3.81; 14 -7.62,3.81
DIL16 = drill 0.813 long: 1 -8.89,-3.81; 2 -6.35,-3.81; 3 -3.81,-3.81; 4 -1.27,-3.81; 5 1.27,-3.81; 6 3.81,-3.81; 7 6.35,-3.81; 8 8.89,-3.81; 9 8.89,3.81; 10 6.35,3.81; 11 3.81,3.81; 12 1.27,3.81; 13 -1.27,3.81; 14 -3.81,3.81; 15 -6.35,3.81; 16 -8.89,3.81
2X3 = drill 1.016 pad 1.88 octagon: 1 0,0; 2 0,2.54; 3 2.54,0; 4 2.54,2.54; 5 5.08,0; 6 5.08,2.54
1X02_LOCK = drill 1.016 pad 1.88: 1 -0.178,0; 2 2.718,0
1X08_LOCK = drill 1.016 pad 1.88 square: 1 0,0.127 | drill 1.016 pad 1.88: 2 2.54,-0.127; 3 5.08,0.127; 4 7.62,-0.127; 5 10.16,0.127; 6 12.7,-0.127; 7 15.24,0.127; 8 17.78,-0.127
2X2 = drill 1.016 pad 1.88 octagon: 1 1.27,3.175; 2 1.27,5.715; 3 3.81,3.175; 4 3.81,5.715
1X03_LOCK = drill 1.016 pad 1.88: 1 0,0.127; 2 2.54,-0.127; 3 5.08,0.127
1X02 = drill 1.016 pad 1.88: 1 0,0; 2 2.54,0
2X10 = drill 1.016 pad 1.88 octagon: 1 -11.43,-1.27; 2 -11.43,1.27; 3 -8.89,-1.27; 4 -8.89,1.27; 5 -6.35,-1.27; 6 -6.35,1.27; 7 -3.81,-1.27; 8 -3.81,1.27; 9 -1.27,-1.27; 10 -1.27,1.27; 11 1.27,-1.27; 12 1.27,1.27; 13 3.81,-1.27; 14 3.81,1.27; 15 6.35,-1.27; 16 6.35,1.27; 17 8.89,-1.27; 18 8.89,1.27; 19 11.43,-1.27; 20 11.43,1.27
2X12 = drill 1.016 pad 1.88 octagon: 1 -13.97,-1.27; 2 -13.97,1.27; 3 -11.43,-1.27; 4 -11.43,1.27; 5 -8.89,-1.27; 6 -8.89,1.27; 7 -6.35,-1.27; 8 -6.35,1.27; 9 -3.81,-1.27; 10 -3.81,1.27; 11 -1.27,-1.27; 12 -1.27,1.27; 13 1.27,-1.27; 14 1.27,1.27; 15 3.81,-1.27; 16 3.81,1.27; 17 6.35,-1.27; 18 6.35,1.27; 19 8.89,-1.27; 20 8.89,1.27; 21 11.43,-1.27; 22 11.43,1.27; 23 13.97,-1.27; 24 13.97,1.27
1X05_LOCK = drill 1.016 pad 1.88: 1 0,0.127; 2 2.54,-0.127; 3 5.08,0.127; 4 7.62,-0.127; 5 10.16,0.127
2X8 = drill 1.016 pad 1.88 octagon: 1 0,0; 2 0,2.54; 3 2.54,0; 4 2.54,2.54; 5 5.08,0; 6 5.08,2.54; 7 7.62,0; 8 7.62,2.54; 9 10.16,0; 10 10.16,2.54; 11 12.7,0; 12 12.7,2.54; 13 15.24,0; 14 15.24,2.54; 15 17.78,0; 16 17.78,2.54
1X04_LOCK = drill 1.016 pad 1.88 square: 1 0,0.127 | drill 1.016 pad 1.88: 2 2.54,-0.127; 3 5.08,0.127; 4 7.62,-0.127
2X4 = drill 1.016 pad 1.88 octagon: 1 -3.81,-1.27; 2 -3.81,1.27; 3 -1.27,-1.27; 4 -1.27,1.27; 5 1.27,-1.27; 6 1.27,1.27; 7 3.81,-1.27; 8 3.81,1.27
POWER_JACK_PTH = drill 2.997 pad 4.318: GND 0,7.7; GNDBREAK 4.7,10.7; PWR 0,13.7
PAD-JUMPER-2-NC_BY_TRACE_YES_SILK = smd 0.635 x 1.27: 1 -0.508,0; 2 0.508,0
LED3MM = drill 0.813 pad 1.676 octagon: A -1.27,0; K 1.27,0
0207/10 = drill 0.813 pad 1.676 octagon: 1 -5.08,0; 2 5.08,0
3RP/1610G = drill 1.2 pad 2.184: 1-1 -5,0; 1-2 0,0; 1-3 5,0; 2-1 -5,5; 2-2 0,5; 2-3 5,5
SIL9 = drill 0.813 long: 1 -10.16,0; 2 -7.62,0; 3 -5.08,0; 4 -2.54,0; 5 0,0; 6 2.54,0; 7 5.08,0; 8 7.62,0; 9 10.16,0
ALPS_POT_ELCON = drill 1.1 pad 1.93: P$1 7,-2.5; P$2 7,0; P$3 7,2.5 | drill 2: P$4 0,-4.4; P$5 0,4.4
TACTILE-PTH = drill 1.016 pad 1.88: 1 -3.251,2.261; 2 3.251,2.261; 3 -3.251,-2.261; 4 3.251,-2.261
DIP08 = drill 0.813 pad 1.727 octagon: 1 -3.81,-3.81; 2 -1.27,-3.81; 3 1.27,-3.81; 4 3.81,-3.81; 5 3.81,3.81; 6 1.27,3.81; 7 -1.27,3.81; 8 -3.81,3.81
1503_09 = drill 0.8 pad 1.2 long: 1 0,-2.1; 2 -4.55,-5.4; 3 5.05,-9.9; 4 -4,-13.1; 5 2.65,-8.5

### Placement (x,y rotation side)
C1  35.56,67.31 90 top
C2  22.86,46.99 270 top
C3  29.21,67.31 90 top
C4  29.21,46.99 270 top
C5  22.86,67.31 90 top
C6  35.56,46.99 270 top
C7  120.02,19.05 180 top
C8  127.64,19.05 180 top
C9  17.78,58.42 270 top
C10  62.87,38.73 270 top
C11  81.28,91.44 90 top
C12  82.55,59.69 90 top
C13  6.35,6.35 90 top
C14  119.38,39.37 270 top
C15  87.63,13.97 90 top
C18  17.14,64.14 180 top
C19  147.32,43.18 270 top
C20  142.24,44.45 270 top
C21  127,91.44 180 top
C22  134.62,83.82 0 top
C23  134.62,88.27 0 top
C24  134.62,79.38 180 top
C25  134.62,74.93 0 top
C26  133.35,70.48 0 top
C27  125.73,70.48 180 top
D1  35.56,81.28 180 top
D2  35.56,34.29 180 top
D3  35.56,31.75 180 top
D4  35.56,78.74 180 top
D5  35.56,76.2 180 top
D6  35.56,29.21 180 top
D11  113.03,64.14 90 top
D12  110.49,64.14 90 top
D13  107.95,64.14 90 top
D14  105.41,64.14 90 top
D15  128.27,99.06 0 top
D16  129.54,61.59 270 top
D17  132.72,61.59 270 top
IC1  29.21,57.15 180 top
IC2  69.85,92.71 180 top
IC3  130.81,38.73 0 top
IC4  75.56,37.47 180 top
IC5  19.05,7.62 180 top
IC6  69.85,60.96 180 top
IC7  74.93,15.24 180 top
J1  43.18,63.5 270 top
J2  77.47,100.97 0 top
J3  59.05,100.97 0 top
J5  71.75,100.97 180 top
J6  61.59,84.45 180 top
J7  77.47,84.45 180 top
J8  67.31,83.82 0 top
J9  109.86,31.11 90 top
J10  115.57,26.04 0 top
J12  119.38,51.44 270 top
J13  129.54,51.44 270 top
J14  43.18,8.89 90 top
J15  93.34,40.64 270 top
J16  20.95,19.05 180 top
J17  77.47,47.62 180 top
J18  96.52,71.12 180 top
J19  78.11,73.66 180 top
J22  105.41,71.75 0 top
J23  105.41,55.88 0 top
J24  92.71,88.9 270 top
J25  105.41,38.1 180 top
J26  99.06,88.9 270 top
J27  105.41,32.38 180 top
J28  105.41,88.9 270 top
J29  126.36,80.01 270 top
J30  96.52,102.23 270 top
J33  21.59,81.28 270 top
J34  21.59,34.29 270 top
J35  43.18,54.61 270 top
J36  45.72,81.28 270 top
J37  44.45,34.29 270 top
J38  91.44,7.62 270 top
J39  92.08,17.14 90 top
J40  72.39,26.67 180 top
J41  72.39,5.71 180 top
J55  86.36,23.5 180 top
J56  81.28,3.81 0 top
J57  105.41,51.44 180 top
J58  105.41,45.09 180 top
J59  146.05,53.34 0 top
J60  139.7,106.05 180 top
J61  128.91,102.23 180 top
JP1  139.7,20.95 180 bottom
LED1  114.3,88.9 0 top
LED2  114.3,93.34 0 top
LED3  114.3,97.79 0 top
LED4  114.3,102.23 0 top
R1  33.66,8.26 270 top
R2  57.15,37.47 270 top
R3  36.2,8.26 270 top
R4  38.73,8.26 270 top
R5  86.36,61.59 90 top
R6  88.9,61.59 90 top
R7  91.44,61.59 90 top
R8  93.98,61.59 90 top
R9  97.79,12.7 180 top
R10  102.87,64.14 270 top
R11  105.41,92.71 180 top
R12  105.41,95.89 180 top
R13  105.41,99.06 180 top
R14  105.41,102.23 180 top
R15  59.69,8.89 90 top
R16  59.69,21.59 90 top
R17  62.23,21.59 270 top
R18  62.23,8.89 90 top
R19  97.79,26.67 0 top
R20  144.78,49.53 180 top
R21  142.88,7.62 270 top
R22  145.41,7.62 90 top
R23  146.69,78.74 90 top
R24  125.73,60.96 270 top
R25  121.92,60.96 90 top
R26  137.79,7.62 90 top
R27  140.34,7.62 90 top
RN1  114.3,42.55 90 top
RN2  128.91,31.11 0 top
RV1  46.61,93.98 90 top
RV2  27.56,93.98 90 top
RV3  8.29,93.98 90 top
RV4  8.29,72.39 90 top
RV5  8.07,50.8 90 top
RV6  8.07,30.48 90 top
RV7  116.2,6.35 90 top
RV8  130.18,6.35 90 top
RV9  144.78,62.23 180 top
S1  100.33,20.32 0 top
S2  100.33,6.35 0 top
U1  146.05,34.29 90 top
X1  151.76,21.59 270 top

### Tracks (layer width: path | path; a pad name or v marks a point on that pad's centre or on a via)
GND
  Top 0.61: U1.4 148.59,38.1 147.32,36.83 | 147.32,36.83 147.32,34.29 148.59,33.02 U1.2 | IC3.7 138.43,38.1 140.97,40.64 142.88,40.64 146.69,36.83 147.32,36.83 | IC7.8 60.96,19.05 59.69,17.78 R16.1
  Top 0.813: C18.2 C5.2
  pour Bottom (isolate 0.305): 0,0 0,106.68 152.4,106.68 152.4,0
N$1
  Top 0.406: D1.C J36.1 J36.2
N$2
  Top 0.406: J36.4 J36.3 D4.C
N$3
  Top 0.406: D5.C J36.5 J36.6
N$4
  Top 0.406: D2.C J37.1 J37.2
N$5
  Top 0.406: J37.4 J37.3 D3.C
N$6
  Top 0.406: D6.C J37.5 J37.6
N$7
  Top 0.406: RN1.1 116.2,32.38 118.11,34.29 122.56,34.29 IC3.1
  Top 0.61: RV7.P$1 118.7,13.38 113.67,18.41 113.67,31.11 RN1.1
N$8
  Top 0.61: RV7.P$2 RV7.P$3 113.68,13.35
  Bottom 0.61: RV7.P$3 113.67,13.39 113.67,13.97 C7.1 114.94,22.86 113.03,22.86 111.76,24.13 111.76,27.3 116.2,31.75 116.2,33.66 117.47,34.92 120.65,34.92 123.19,37.47 IC3.2
N$9
  Top 0.406: RN2.1 118.75,32.38 119.38,33.02 126.36,33.02 IC3.3
  Bottom 0.61: RV8.P$1 135.89,16.57 135.89,26.67 137.79,28.57 139.7,28.57 140.34,29.21 140.34,36.83 138.43,38.73 128.27,38.73 IC3.3
N$10
  Bottom 0.61: RV8.P$2 RV8.P$3 126.36,14.66 C8.1 121.28,24.13 114.3,24.13 113.03,25.4 113.03,26.67 117.47,31.11 117.47,32.38 118.11,33.02 129.54,33.02 130.81,34.29 IC3.4
N$11
  Top 0.406: J12.3 J12.4 126.36,47.62 129.54,44.45 129.54,40.64 133.35,36.83 IC3.5
N$12
  Top 0.406: J39.2 100.33,19.68 101.6,18.41 101.6,13.97 R9.1
N$13
  Bottom 0.406: JP1.1 138.66,21.48 X1.4
N$15
  Bottom 0.61: C20.1 142.24,46.99 R20.2
N$16
  Top 0.406: C19.1 146.05,43.18 C20.2
  Bottom 0.61: C20.2 U1.5
N$17
  Top 1.27: J60.PWR 138.79,91.44 133.35,91.44 130.81,93.98 130.81,98.42 131.44,99.06 | 131.44,99.06 D15.A | J61.1 131.44,99.69 131.44,99.06
N$19
  Top 0.406: J35.2 J35.1 41.27,56.52 24.77,56.52 IC1.8 17.14,53.34 15.24,55.24 15.24,59.69 7.62,67.31 7.62,77.56 RV4.P$3
N$20
  Top 0.406: LED4.A R14.1
N$23
  Top 0.406: J27.1 105.16,32.51 J27.2 102.62,32.26 J27.3 100.08,32.51 J27.4
N$24
  Top 0.406: J28.1 105.28,88.65 J28.2 105.54,86.11 J28.3 105.28,83.57 J28.4
N$25
  Top 0.406: LED3.A 111.76,99.06 R13.1
N$26
  Top 0.406: R12.1 LED2.A
N$27
  Top 0.406: R11.1 113.03,90.17 LED1.A
N$28
  Top 0.61: R21.2 138.43,6.99 138.43,9.53 135.89,12.06 135.89,17.14 133.99,19.05 C8.2
N$30
  Top 0.406: J30.1 R14.2
N$31
  Top 0.406: J1.4 J1.3 41.27,59.05 30.48,59.05 29.21,60.33 IC1.4 29.21,62.23 31.75,64.77 31.75,71.12 34.29,73.66 34.29,100.33 31.75,102.87 26.95,102.87 RV2.P$3
N$32
  Top 0.406: J35.4 J35.3 40.01,55.24 27.94,55.24 26.67,53.98 IC1.10 24.77,51.44 17.14,51.44 13.97,54.61 8.76,54.61 RV5.P$3
N$33
  Top 0.406: J1.6 J1.5 42.55,57.78 29.84,57.78 28.57,59.05 24.77,59.05 24.13,59.69 IC1.6
  Bottom 0.406: RV3.P$3 10.16,96.61 10.16,83.82 20.32,73.66 20.32,66.04 24.13,62.23 IC1.6
N$34
  Bottom 0.406: J2.2 77.47,98.25 IC2.1
N$35
  Bottom 0.406: J2.1 74.93,98.6 IC2.2
N$36
  Bottom 0.406: J3.2 63.68,99.06 66.04,99.06 67.31,97.79 IC2.5
N$37
  Bottom 0.406: J3.1 60.78,99.06 62.23,99.06 IC2.6
N$38
  Bottom 0.406: IC2.8 58.42,85.09 58.42,83.82 58.88,84.28 J6.2
N$39
  Bottom 0.406: IC2.9 61.77,85.9 J6.1
N$40
  Bottom 0.406: IC2.12 74.75,86.54 J7.2
N$41
  Bottom 0.406: IC2.13 77.65,86.18 J7.1
N$42
  Bottom 0.406: IC2.11 70.03,88.72 J8.2
N$43
  Bottom 0.406: IC2.10 67.13,88.72 J8.1
N$44
  Bottom 0.406: J5.2 69.85,100.15 IC2.4
N$45
  Bottom 0.406: J5.1 72.39,100.51 IC2.3
N$46
  Top 0.406: IC6.9 66.04,52.07 95.25,52.07 97.79,54.61 97.79,64.77 95.89,66.67 R8.2
  Bottom 0.406: J18.1 94.04,68.52 | 94.04,68.52 93.98,68.45 | R8.2 94.04,66.74 94.04,68.52
N$47
  Top 0.406: IC6.10 67.31,53.34 93.98,53.34 96.52,55.88 96.52,62.23 95.25,63.5 92.71,63.5 91.44,64.77 R7.2
  Bottom 0.406: J18.2 91.44,68.71 R7.2
N$48
  Top 0.406: IC6.11 68.58,54.61 81.92,54.61 88.9,61.59 R6.2
  Bottom 0.406: J18.3 88.9,68.45 R6.2
N$49
  Top 0.406: IC6.6 64.77,66.04 64.77,67.31 63.5,68.58 59.69,68.58 58.42,69.85 58.42,76.2 61.59,79.38 83.19,79.38 88.9,74.93 J18.4
  Bottom 0.406: J18.4 86.36,68.71 R5.2
N$51
  Top 0.406: J19.2 80.01,69.22 80.01,62.23 78.74,60.96 74.3,60.96 71.12,57.78 IC6.13
  Bottom 0.406: J19.1 J19.2
N$52
  Top 0.406: J19.4 J19.3 75.56,76.2 76.2,76.83 80.64,76.83 81.92,75.56 81.92,65.41 81.28,64.77 81.28,61.59 79.38,59.69 74.93,59.69 73.66,58.42 IC6.14
  Bottom 0.406: J19.3 J19.4
N$53
  Top 0.406: J19.6 73.03,75.56 75.56,78.11 81.28,78.11 83.19,76.2 83.19,65.41 84.45,64.14 84.45,59.05 80.64,55.24 77.47,55.24 76.2,56.52 IC6.15
  Bottom 0.406: J19.5 J19.6
N$54
  Top 0.406: J19.8 69.85,70.48 69.85,60.33 68.58,59.05 IC6.12
  Bottom 0.406: J19.7 J19.8
N$55
  Bottom 0.406: J19.10 J19.9 69.85,75.56 79.38,75.56 80.64,74.3 80.64,66.04 79.38,64.77 IC6.1
N$56
  Top 0.406: J19.12 68.58,67.94 IC6.5
  Bottom 0.406: J19.11 J19.12
N$57
  Bottom 0.406: J19.13 J19.14 65.41,68.58 73.66,68.58 76.2,66.04 IC6.2
N$58
  Bottom 0.406: J19.15 J19.16 64.14,67.31 68.58,67.31 IC6.4
N$59
  Bottom 0.406: J18.5 81.92,67.82 81.92,64.77 79.38,62.23 75.56,62.23 73.66,64.14 IC6.3
N$60
  Top 0.406: J15.1 91.44,38.73 91.44,34.29 88.27,31.11 73.03,31.11 72.39,31.75 72.39,33.02 IC4.11 69.85,35.56 66.04,35.56 62.87,32.38 R2.2
N$61
  Bottom 0.406: IC4.10 71.12,31.75 90.17,31.75 93.34,34.92 J15.2
N$62
  Top 0.406: IC4.9 67.31,33.02 67.31,31.75 68.58,30.48 90.17,30.48 95.25,35.56 95.25,42.55 J17.2 J17.1
N$63
  Top 0.406: J17.3 J17.4
  Bottom 0.406: J17.4 88.9,40.01 85.72,36.83 73.66,36.83 IC4.7
N$64
  Top 0.406: J17.5 J17.6
  Bottom 0.406: J17.6 86.36,45.09 87,44.45 87,40.01 85.09,38.1 74.93,38.1 IC4.6
N$65
  Top 0.406: J17.7 J17.8
  Bottom 0.406: J17.8 83.82,45.09 85.72,43.18 85.72,40.01 85.09,39.37 74.93,39.37 74.3,40.01 IC4.5
N$66
  Top 0.406: J17.9 J17.10
  Bottom 0.406: J17.10 81.28,45.09 79.38,43.18 IC4.3
N$67
  Top 0.406: J17.11 J17.12 78.74,45.72 81.92,42.55 IC4.2
N$68
  Top 0.406: J17.13 J17.14 76.2,43.81 76.83,43.18 IC4.4
N$69
  Top 0.406: J17.15 J17.16 73.66,44.45 75.56,42.55 75.56,36.83 76.83,35.56 IC4.13
N$70
  Top 0.406: J17.17 J17.18 71.12,45.09 73.03,43.18 73.03,37.47 74.3,36.2 IC4.12
N$71
  Top 0.406: J17.19 J17.20 68.58,45.09 70.48,43.18 70.48,39.37 71.75,38.1 71.75,36.83 73.03,35.56 73.03,32.38 73.66,31.75 78.11,31.75 78.74,32.38 78.74,33.02 IC4.14
N$72
  Top 0.406: J17.21 J17.22
  Bottom 0.406: J17.22 66.04,45.09 67.94,43.18 67.94,38.1 70.48,35.56 81.28,35.56 81.92,34.92 IC4.15
N$73
  Top 0.254: 82.55,43.18 82.55,50.16
  Top 0.406: J17.24 J17.23 63.5,49.53 64.77,50.8 81.92,50.8 82.55,50.16 | IC4.1 82.55,43.18
N$74
  Top 0.406: R4.2 38.73,4.57 J14.1
  Bottom 0.406: IC5.15 25.4,5.08 27.94,7.62 35.56,7.62 38.73,4.45 R4.2
N$75
  Top 0.406: R3.2 36.2,4.32 J14.2
  Bottom 0.406: IC5.13 22.23,1.91 34.92,1.91 R3.2
N$76
  Top 0.406: R1.2 33.66,4.57 | 33.66,4.57 J14.3 | 33.66,4.57 30.99,1.91 24.13,1.91 22.86,3.17 IC5.14
N$77
  Bottom 0.406: J16.1 J16.2 32.38,17.14 29.21,13.97 24.13,13.97 22.86,12.7 IC5.3
N$78
  Top 0.406: IC5.2 25.4,12.7 29.21,16.51 29.21,17.14 J16.4
  Bottom 0.406: J16.3 J16.4
N$79
  Bottom 0.406: J16.5 J16.6 27.3,17.14 25.4,15.24 22.86,15.24 20.32,12.7 IC5.4
N$80
  Top 0.406: IC5.7 12.7,12.7 13.97,13.97 22.86,13.97 24.13,15.24 24.13,17.14 J16.8
  Bottom 0.406: J16.7 J16.8
N$81
  Bottom 0.406: J16.9 J16.10 22.23,17.14 19.05,13.97 19.05,8.89 17.78,7.62 16.51,7.62 IC5.10
N$82
  Top 0.406: IC5.1 29.21,11.43 34.29,16.51 34.29,21.59 33.02,22.86 21.59,22.86 20.32,21.59 20.32,20.95 J16.11
  Bottom 0.406: J16.11 J16.12
N$83
  Bottom 0.406: J16.13 J16.14 17.14,12.06 IC5.5
N$84
  Bottom 0.406: J16.15 J16.16 14.61,12.06 IC5.6
N$85
  Bottom 0.406: J16.17 J16.18 12.06,17.14 8.89,13.97 8.89,5.08 IC5.9
N$86
  Top 0.406: J16.20 9.53,14.61 8.89,13.97 8.89,8.89 10.16,7.62 12.7,7.62 15.24,5.08 IC5.11
  Bottom 0.406: J16.19 J16.20
N$87
  Top 0.406: J12.1 J12.2 127,50.16 131.44,45.72 133.99,45.72 135.89,43.81 IC3.9
N$88
  Bottom 0.61: X1.3 141.87,14.23 R27.2 140.34,6.35 137.79,3.81 R26.1
N$89
  Top 0.406: J35.6 J35.5 41.91,50.8 33.02,50.8 31.75,52.07 | IC1.12 31.75,52.7 31.75,52.07 | RV6.P$3 17.62,49.53 29.21,49.53 31.75,52.07
N$90
  Bottom 0.406: J29.2 126.36,72.39 C27.2
N$91
  Top 0.406: J30.2 97.03,99.06 R13.2
N$92
  Top 0.406: R25.1 R24.2 128.27,58.42 128.27,60.96 130.81,63.5 130.81,67.31 133.35,67.31 134.62,68.58 C26.2
  Bottom 0.61: IC3.13 124.46,43.81 124.46,44.45 123.19,45.72 121.28,45.72 120.02,46.99 120.02,54.61 121.28,55.88 R25.1
N$93
  Top 0.406: J30.3 97.92,95.89 R12.2
N$94
  Top 0.406: J30.4 98.3,92.71 R11.2
N$95
  Top 0.406: RN2.9 133.35,25.4 J10.8
N$96
  Top 0.406: RN2.8 132.72,27.3 131.95,27.3 J10.7
N$97
  Top 0.406: R15.2 59.69,8.89 65.41,3.17 66.04,3.17 66.67,2.54 79.88,2.54 J56.1
  Bottom 0.406: J56.1 81.28,7.62 78.74,10.16 IC7.14
N$98
  Top 0.406: R16.2 63.5,22.86 67.31,22.86 68.58,21.59 69.85,21.59 71.12,20.32 IC7.6 71.12,18.41 72.39,17.14 85.09,17.14 86.36,18.41 J55.1
N$99
  Top 0.406: RN2.7 131.44,28.57 130.81,28.57 130.18,27.94 128.91,27.94 128.27,27.3 J10.6
N$100
  Top 0.406: RN2.6 131.44,30.48 129.54,28.57 128.14,28.57 J10.5
N$101
  Top 0.406: RN2.5 128.91,30.48 126.36,27.94 124.46,27.94 123.83,27.3 123.83,26.54 J10.4
N$102
  Top 0.406: RN2.4 123.19,27.94 122.43,27.94 J10.3
N$103
  Top 0.406: RN2.3 120.65,27.94 119.38,27.94 118.11,26.67 J10.2
N$104
  Top 0.406: RN2.2 118.11,27.94 116.84,27.94 115.57,26.67 J10.1
N$105
  Top 0.406: J9.8 110.62,50.93 111.76,52.07 114.3,52.07 RN1.9
N$106
  Top 0.406: J9.7 110.49,45.72 112.39,47.62 112.39,48.9 113.03,49.53 114.3,49.53 RN1.8
N$107
  Top 0.406: J9.6 110.62,43.94 113.03,46.35 113.67,46.35 RN1.7
N$108
  Top 0.406: J9.5 110.49,40.64 RN1.6
N$109
  Top 0.406: J9.4 110.62,38.23 RN1.5
N$110
  Top 0.406: J9.3 110.49,35.56 RN1.4
N$111
  Top 0.406: J9.2 110.62,33.15 RN1.3
N$112
  Top 0.406: J9.1 110.49,30.48 RN1.2
N$113
  Top 0.406: J13.3 J13.4 135.25,46.35 137.16,44.45 137.16,36.2 IC3.6
N$115
  Top 0.61: R26.2 137.79,17.78 134.62,20.95 123.19,20.95 C7.2
N$116
  Bottom 0.406: J22.4 D11.A
N$117
  Bottom 0.406: J22.3 D12.A
N$118
  Top 0.406: J13.1 J13.2 138.43,46.99 IC3.8
N$121
  Bottom 0.406: J22.2 D13.A
N$122
  Bottom 0.406: J22.1 D14.A
N$123
  Top 0.406: 109.22,60.33 D13.C D14.C 104.14,60.33 R10.2 | 109.22,60.33 D12.C D11.C | J23.2 J23.1 109.22,59.69 109.22,60.33
N$124
  Bottom 0.406: IC7.9 66.04,15.24 64.77,16.51 R17.2 64.14,18.41 64.14,27.3 67.94,31.11 79.38,31.11 80.64,29.84 80.64,28.57 83.82,25.4 J55.2
N$125
  Top 0.406: J1.2 J1.1 35.56,63.5 34.29,62.23 IC1.2
  Bottom 0.406: RV1.P$3 40.01,96.88 40.01,91.44 43.18,88.27 J1.1
N$126
  Top 0.406: R17.1 64.77,26.67 68.58,22.86 78.74,22.86 80.01,21.59 82.55,21.59 83.82,20.32 IC7.1
  Bottom 0.406: J56.2 83.95,3.68 85.72,1.91 87.63,1.91 88.9,3.17 88.9,5.08 85.72,8.26 85.72,13.34 83.82,15.24 IC7.1
N$127
  Top 0.406: J33.1 J33.2 D1.A | RV1.P$2 RV1.P$1
  Bottom 0.406: 36.83,60.33 IC1.1 36.83,64.77 C1.1 31.11,70.48 31.11,73.66 29.84,74.93 28.57,74.93 27.3,76.2 27.3,80.01 26.04,81.28 J33.2 | D1.A 38.73,88.27 38.73,103.5 40.01,104.78 45.09,104.78 46.61,103.25 RV1.P$2
N$128
  Top 0.406: J25.4 98.04,37.97 J25.3 100.46,38.1 102.87,38.1 J25.2 103.12,37.97 J25.1
N$130
  Bottom 0.61: C19.2 147.32,51.89 J59.1
N$131
  Top 0.406: D4.A J33.4 J33.3 | RV2.P$1 RV2.P$2
  Bottom 0.406: IC1.3 31.75,63.5 C3.1 26.04,69.22 26.04,76.83 J33.4 | RV2.P$1 29.21,100.13 29.21,80.01 30.48,78.74 D4.A
N$132
  Top 0.406: J38.1 78.74,7.62 77.47,8.89 69.85,8.89 68.58,10.16 IC7.10
  Bottom 0.406: J40.7 J40.8 68.58,22.86 67.31,21.59 | 67.31,21.59 67.31,12.7 | 67.31,12.7 IC7.10 | 67.31,21.59 67.31,12.7
N$133
  Top 0.406: R18.2 80.01,13.97 81.28,12.7 IC7.15
  Bottom 0.406: IC7.15 81.28,10.16 85.09,6.35 85.09,5.21 J56.3
N$134
  Top 0.406: J38.2 91.31,4.95 88.27,1.91 64.14,1.91 R18.1
N$135
  Bottom 0.406: J41.8 J41.7 68.58,8.89 69.85,10.16 69.85,13.34 71.12,14.61 76.83,14.61 IC7.2 81.28,19.68 82.55,20.95 88.27,20.95 91.95,17.27 J39.1
N$136
  Top 0.406: S1.3 97.08,17.07 R9.2 | IC7.7 71.75,15.88 81.92,15.88 82.55,15.24 82.55,10.16 83.82,8.89 86.36,8.89 89.53,12.06 92.08,12.06 R9.2 | 92.71,12.06 R9.2
  Bottom 0.406: R9.2 92.71,10.79 96.52,6.99 96.52,4.65 S2.3 | S1.3 97.08,19.13 95.25,20.95 95.25,22.86 93.98,24.13 90.81,24.13 88.27,21.59 82.04,21.59 80.77,22.86 J55.3
N$137
  Top 0.406: S1.1 101.17,26.67 R19.2
N$138
  Bottom 0.406: IC7.11 J41.5 J41.6
N$139
  Bottom 0.406: IC7.12 J41.3 J41.4
N$140
  Bottom 0.406: J41.2 J41.1 IC7.13
N$141
  Bottom 0.406: J40.6 J40.5 71.12,29.84 71.75,30.48 78.74,30.48 79.38,29.84 79.38,19.68 IC7.3
N$142
  Bottom 0.406: J40.4 J40.3 73.66,28.57 74.93,29.84 77.47,29.84 78.11,29.21 78.11,21.59 76.2,19.68 IC7.4
N$143
  Bottom 0.406: J40.2 J40.1 76.2,22.86 73.66,20.32 IC7.5
N$144
  Top 0.406: J33.5 J33.6 D5.A | RV3.P$1 RV3.P$2
  Bottom 0.406: IC1.5 26.67,62.23 C5.1 21.59,67.31 J33.5 20.32,76.2 19.05,77.47 19.05,92.72 RV3.P$1
N$145
  Top 0.406: J34.1 J34.2 D2.A | RV4.P$1 RV4.P$2
  Bottom 0.406: J34.2 24.13,34.92 24.77,35.56 24.77,46.35 C2.1 22.86,52.07 IC1.9 21.59,50.8 19.05,50.8 12.7,57.15 12.7,68.58 8.29,72.99 RV4.P$2
N$146
  Top 0.406: D3.A J34.4 J34.3 | RV5.P$1 RV5.P$2 8.07,59.24 6.99,60.33 5.08,60.33 3.17,58.42 3.17,56.52 3.81,55.24 5.71,55.24 7.62,53.34 13.34,53.34 16.51,50.16 26.04,50.16 IC1.11
  Bottom 0.406: IC1.11 C4.1 26.67,45.72 26.67,33.02 25.4,31.75 J34.4
N$147
  Top 0.406: D6.A J34.6 J34.5 18.84,29.21 RV6.P$1 RV6.P$2
  Bottom 0.406: IC1.13 35.56,52.07 C6.1 31.11,43.81 31.11,38.1 27.94,34.92 27.94,31.75 25.4,29.21 J34.6
N$148
  Top 0.406: R21.1 R22.2
  Bottom 0.61: R22.2 145.41,25.19 X1.2
N$151
  Bottom 0.406: JP1.2 140.84,21.59 141.79,21.59
  Bottom 0.61: U1.3 141.79,27.5 141.79,21.59 141.79,21.05 X1.5
N$153
  Bottom 0.406: C27.1 D16.C 130.81,64.14 130.81,59.69 D17.A
N$154
  Bottom 0.406: C24.2 C25.1 133.99,74.3 133.99,73.03 134.62,72.39 136.53,72.39 138.43,70.48 138.43,69.22 134.62,65.41 D17.C | RV9.P$3 135.85,59.73 133.35,62.23
  Bottom 0.61: 133.35,62.23 132.72,62.87 D17.C
N$155
  Top 0.406: R23.2-1 R23.1-2 R23.1-3
  Bottom 0.406: R23.1-3 146.13,83.74 142.24,87.63 136.53,87.63 | 136.53,87.63 C23.2 | 136.53,87.63 136.53,84.45 C22.2
N$156
  Top 0.406: R23.2-3 R23.2-2 | R25.2 121.92,71.12 125.73,74.93 129.54,74.93 132.08,77.47 133.99,77.47 C24.1
  Bottom 0.406: R23.2-2 136.53,78.74 C24.1
  Bottom 0.61: R25.2 127.64,60.33 127.64,55.24 130.81,52.07 130.81,46.35 133.35,43.81 IC3.10
N$157
  Top 0.406: C25.2 139.7,71.12 144.78,71.12 146.69,73.03 R23.1-1
  Bottom 0.61: IC3.11 133.35,40.01 139.06,40.01 139.7,40.64 139.7,46.35 137.79,48.26 137.79,51.44 141.6,55.24 141.6,69.85 145.5,73.74 R23.1-1
N$158
  Top 0.406: R24.1 128.27,68.58 130.18,68.58 C26.1
  Bottom 0.406: J29.1 128.09,80.19 129.54,78.74 129.54,74.93 132.08,71.75 C26.1
  Bottom 0.61: IC3.12 127,43.81 127,52.07 123.83,55.24 123.83,56.52 120.02,60.33 120.02,67.31 121.28,68.58 125.09,68.58 125.73,67.94 R24.1
VCC
  Bottom 0.406: IC4.16 93.98,43.18 93.98,48.26 95.25,49.53 | 95.25,49.53 97.28,51.56 J57.4 | R19.1 95.25,29.21 95.25,49.53
  Bottom 0.61: IC1.14 36.83,57.15 35.56,58.42 C9.1 | C12.1 82.55,57.15 86.36,53.34 96.01,53.34 J57.4
  pour Top: 0,0 0,106.68 152.4,106.68 152.4,0

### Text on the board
tDocu: Out | LED | 5-9V DC | In B | B A | In A | GND | Vcc | 1 | 2 | 3 | 4 | 5-9V DC | OSC C | OSC B | OSC A | 4070 | Input | XOR | Drum | A | In D | D C | In C | Out | In | B | 7 | 6 | 5 | 4 | 3 | 2 | 1 | 0 | Vcc | GND | Mult | C | Out | OR Gate | X | Inh | A | B | C | Sync | In | C | B | A | Mux | Outputs | OSC D | A | 4 / 0 / 5 / 1 | B | C | Out | SPKR | D | Divided / Outs | 12 | 11 | 10 | 9 | 8 | 7 | 6 | 5 | 4 | 3 | 2 | 1 | In | Out | E | Vcc | F | OSC Out | Buffer | OSC E | D | E | F | Gnd | Rst | Clk | 40106 Oscillators | Mult | D | 4040 | Binary counter | E | F | Input | Sync | A | Rst | Dat | Clk | Recirculate | OSC F | Low Gain (left) | 4 | 3 | 2 | 1 | 4017 | Decade Counter | Count | Set | 9 | 8 | 7 | 6 | 5 | 4 | 3 | 2 | 1 | 0 | Clock | Inhibit | 4 / 0 / 1 / 5 | 8 Stage | Reset | High Gain (Right) | R | D | C | 100nF | B | 4 | 3 | 2 | 1 | Clear
bDocu: Logic: / Elliot Williams / https://hackaday.com/tag/logic-noise | Layout: / Avik D / avik.tk@gmail.com

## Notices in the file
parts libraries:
SparkFun-Aesthetics: Licensing: Creative Commons ShareAlike 4.0 International - https://creativecommons.org/licenses/by-sa/4.0
